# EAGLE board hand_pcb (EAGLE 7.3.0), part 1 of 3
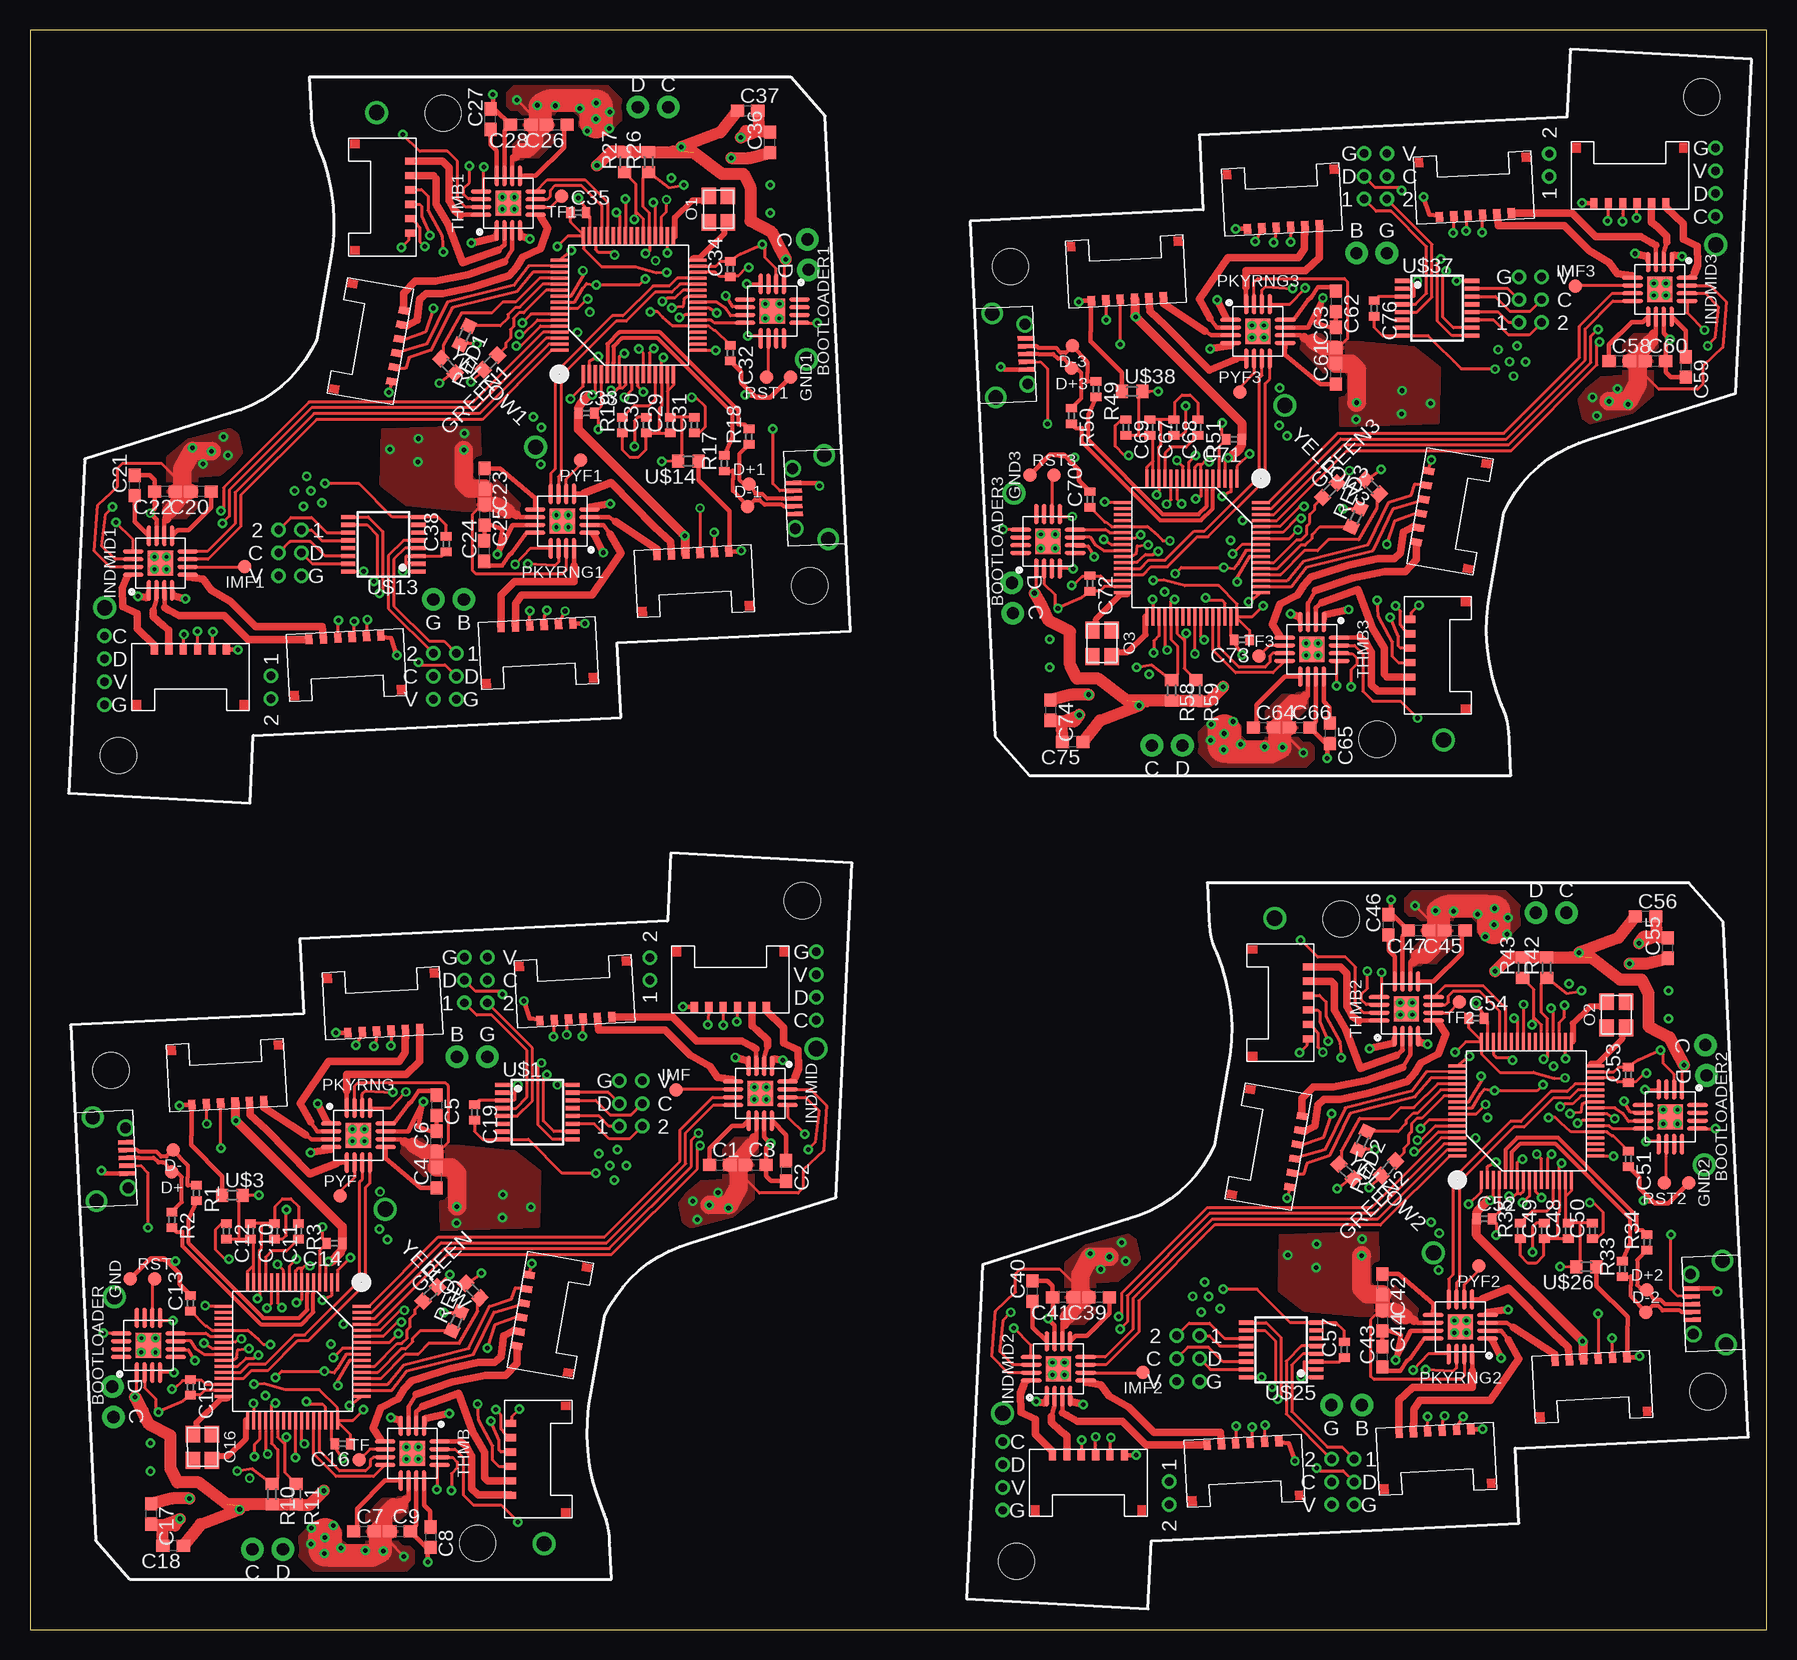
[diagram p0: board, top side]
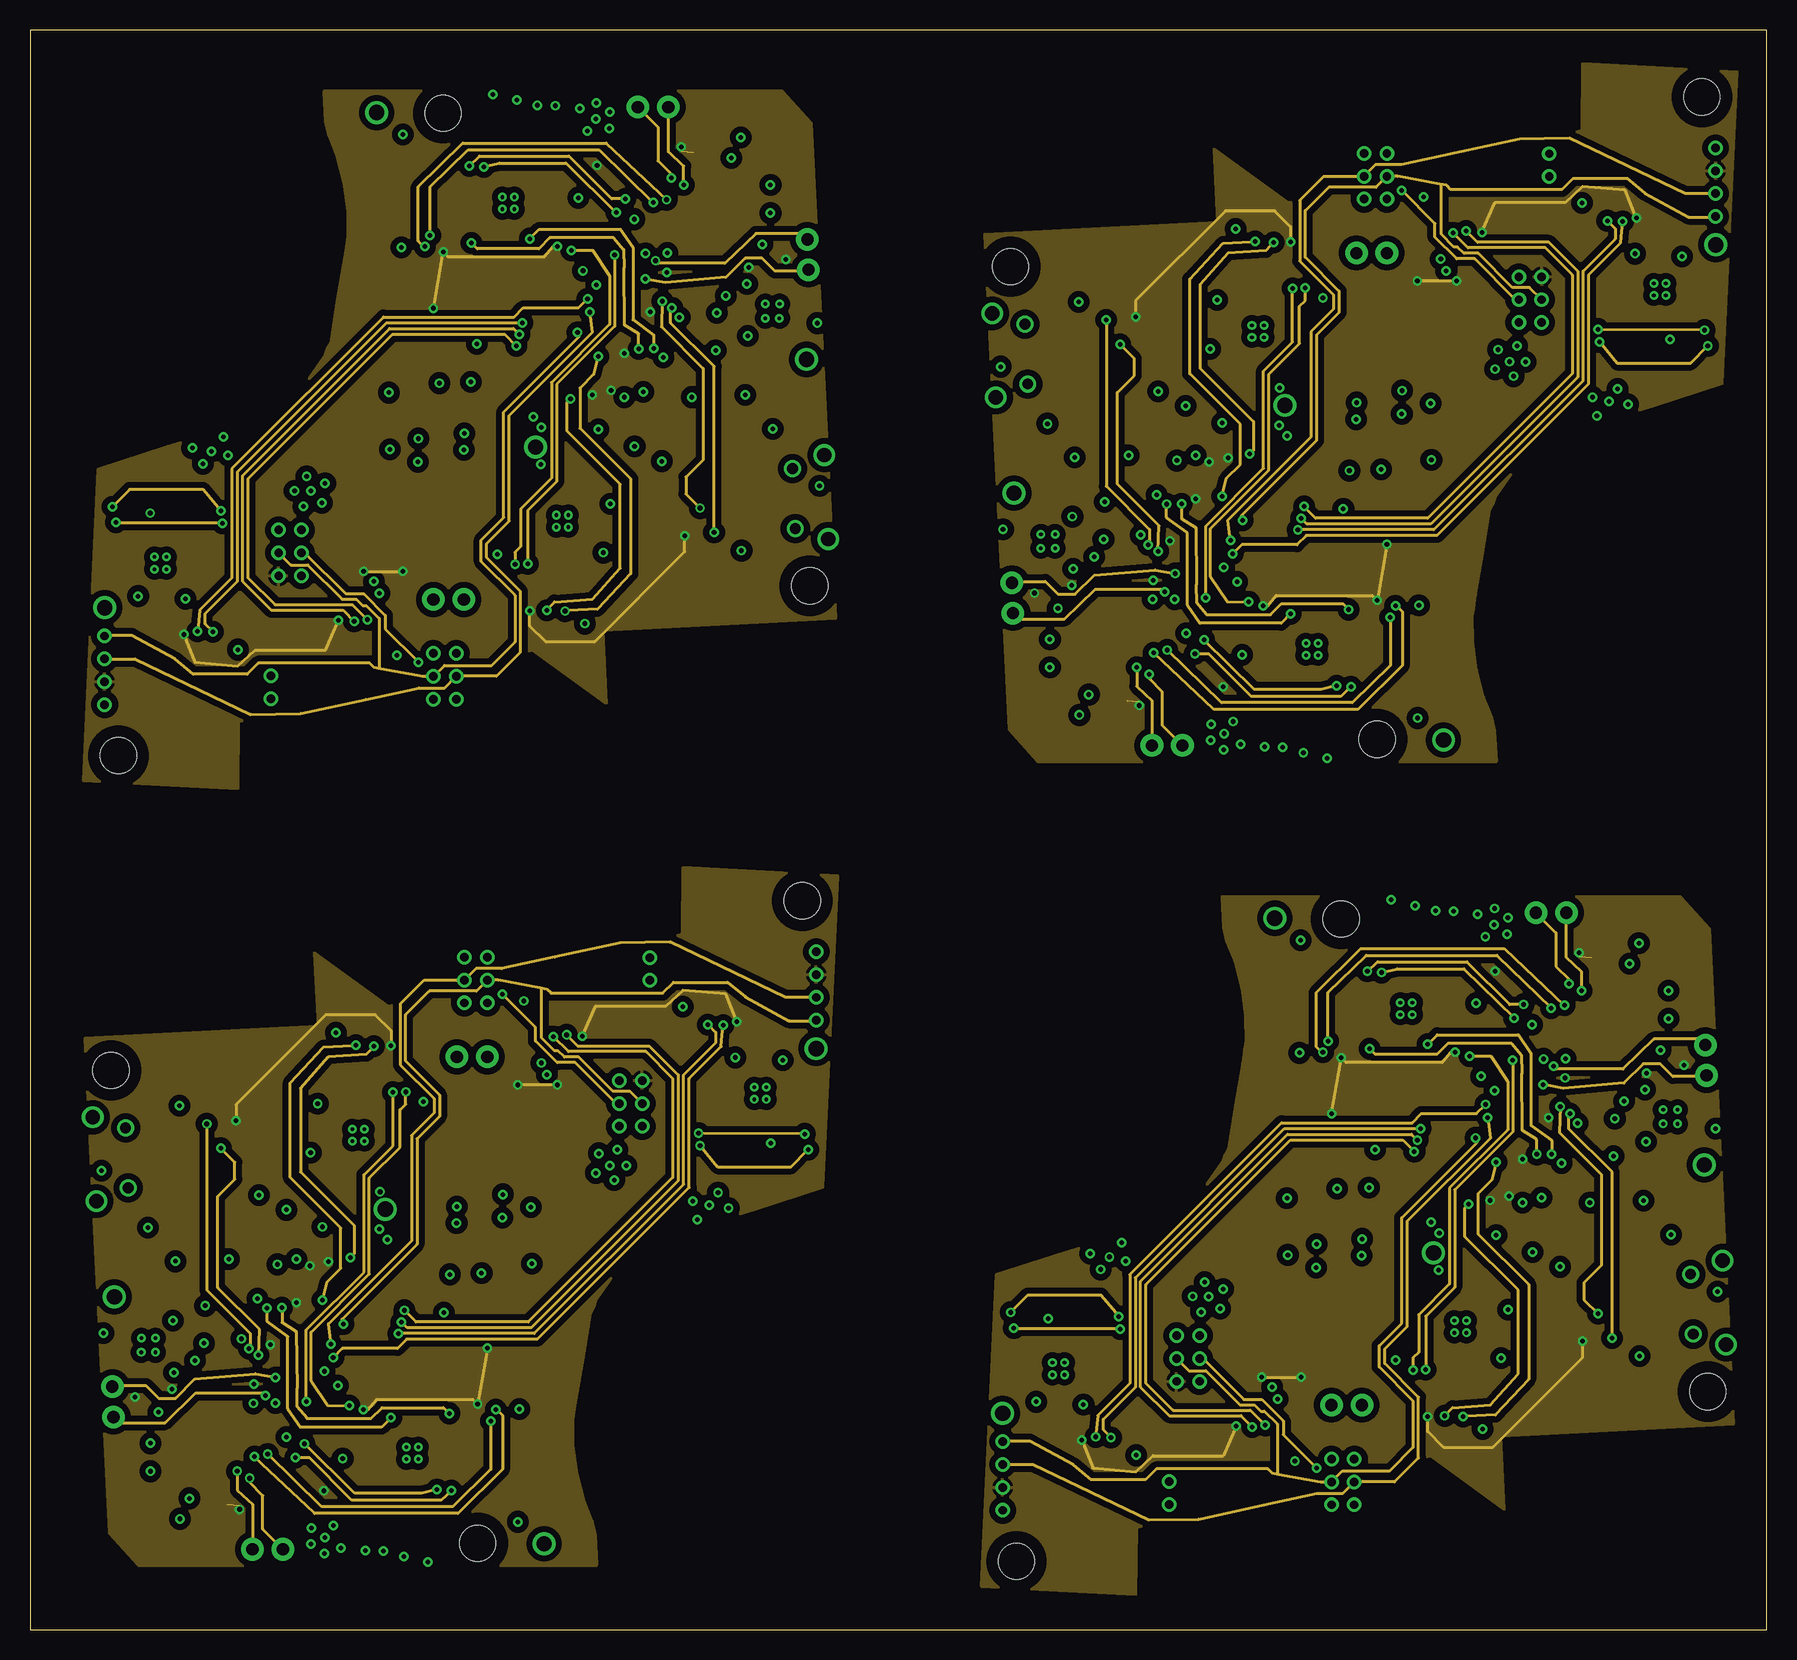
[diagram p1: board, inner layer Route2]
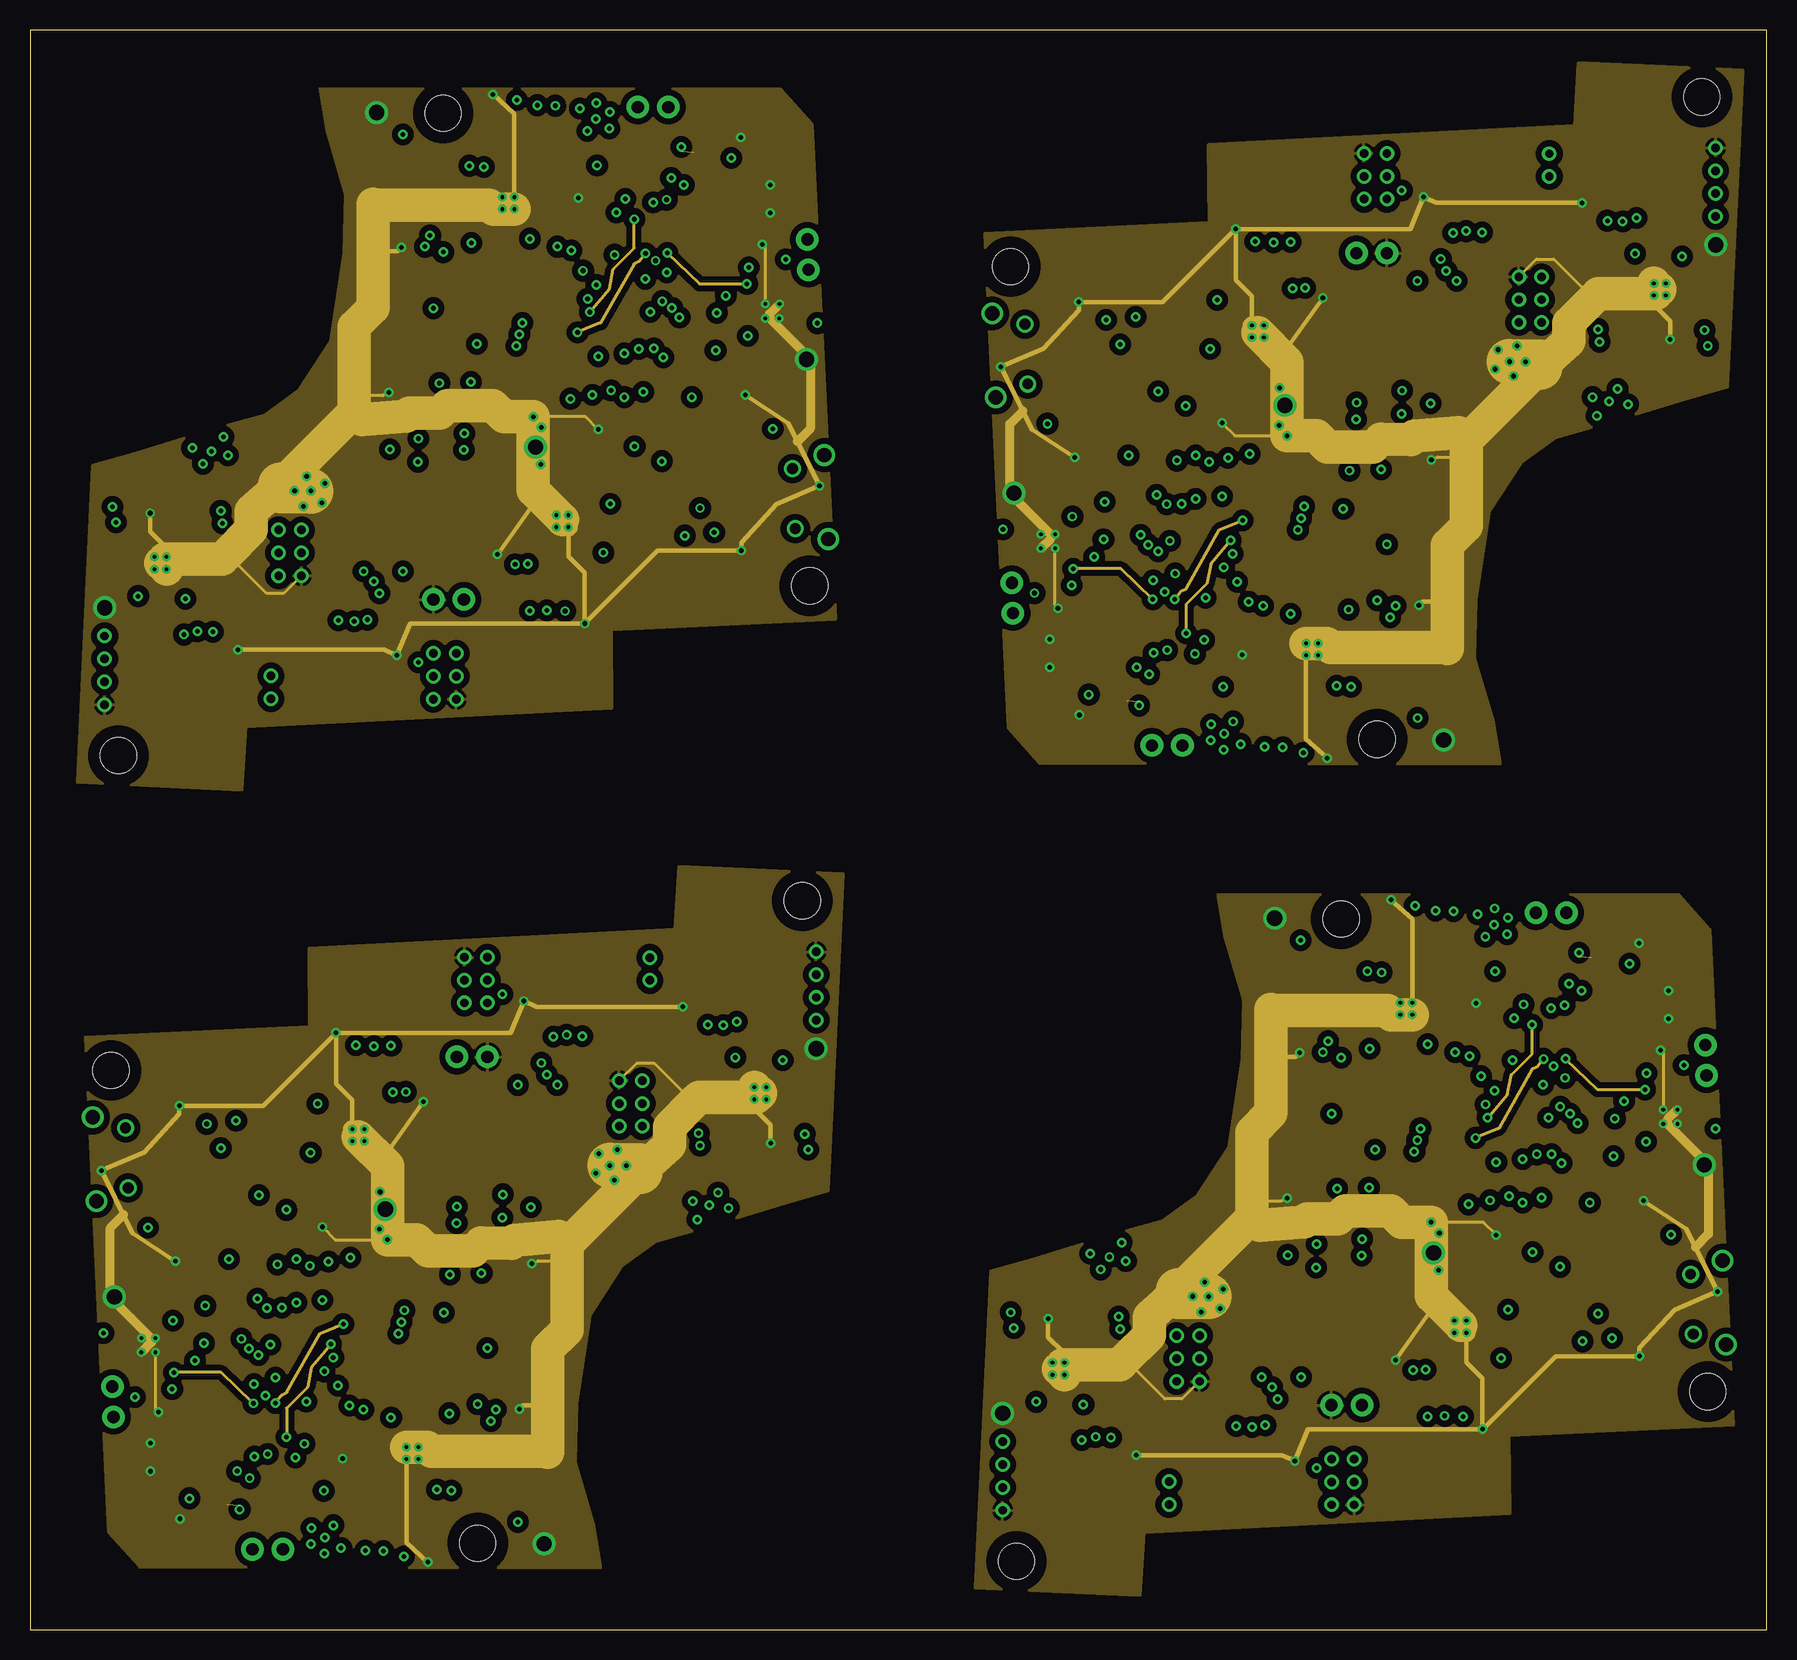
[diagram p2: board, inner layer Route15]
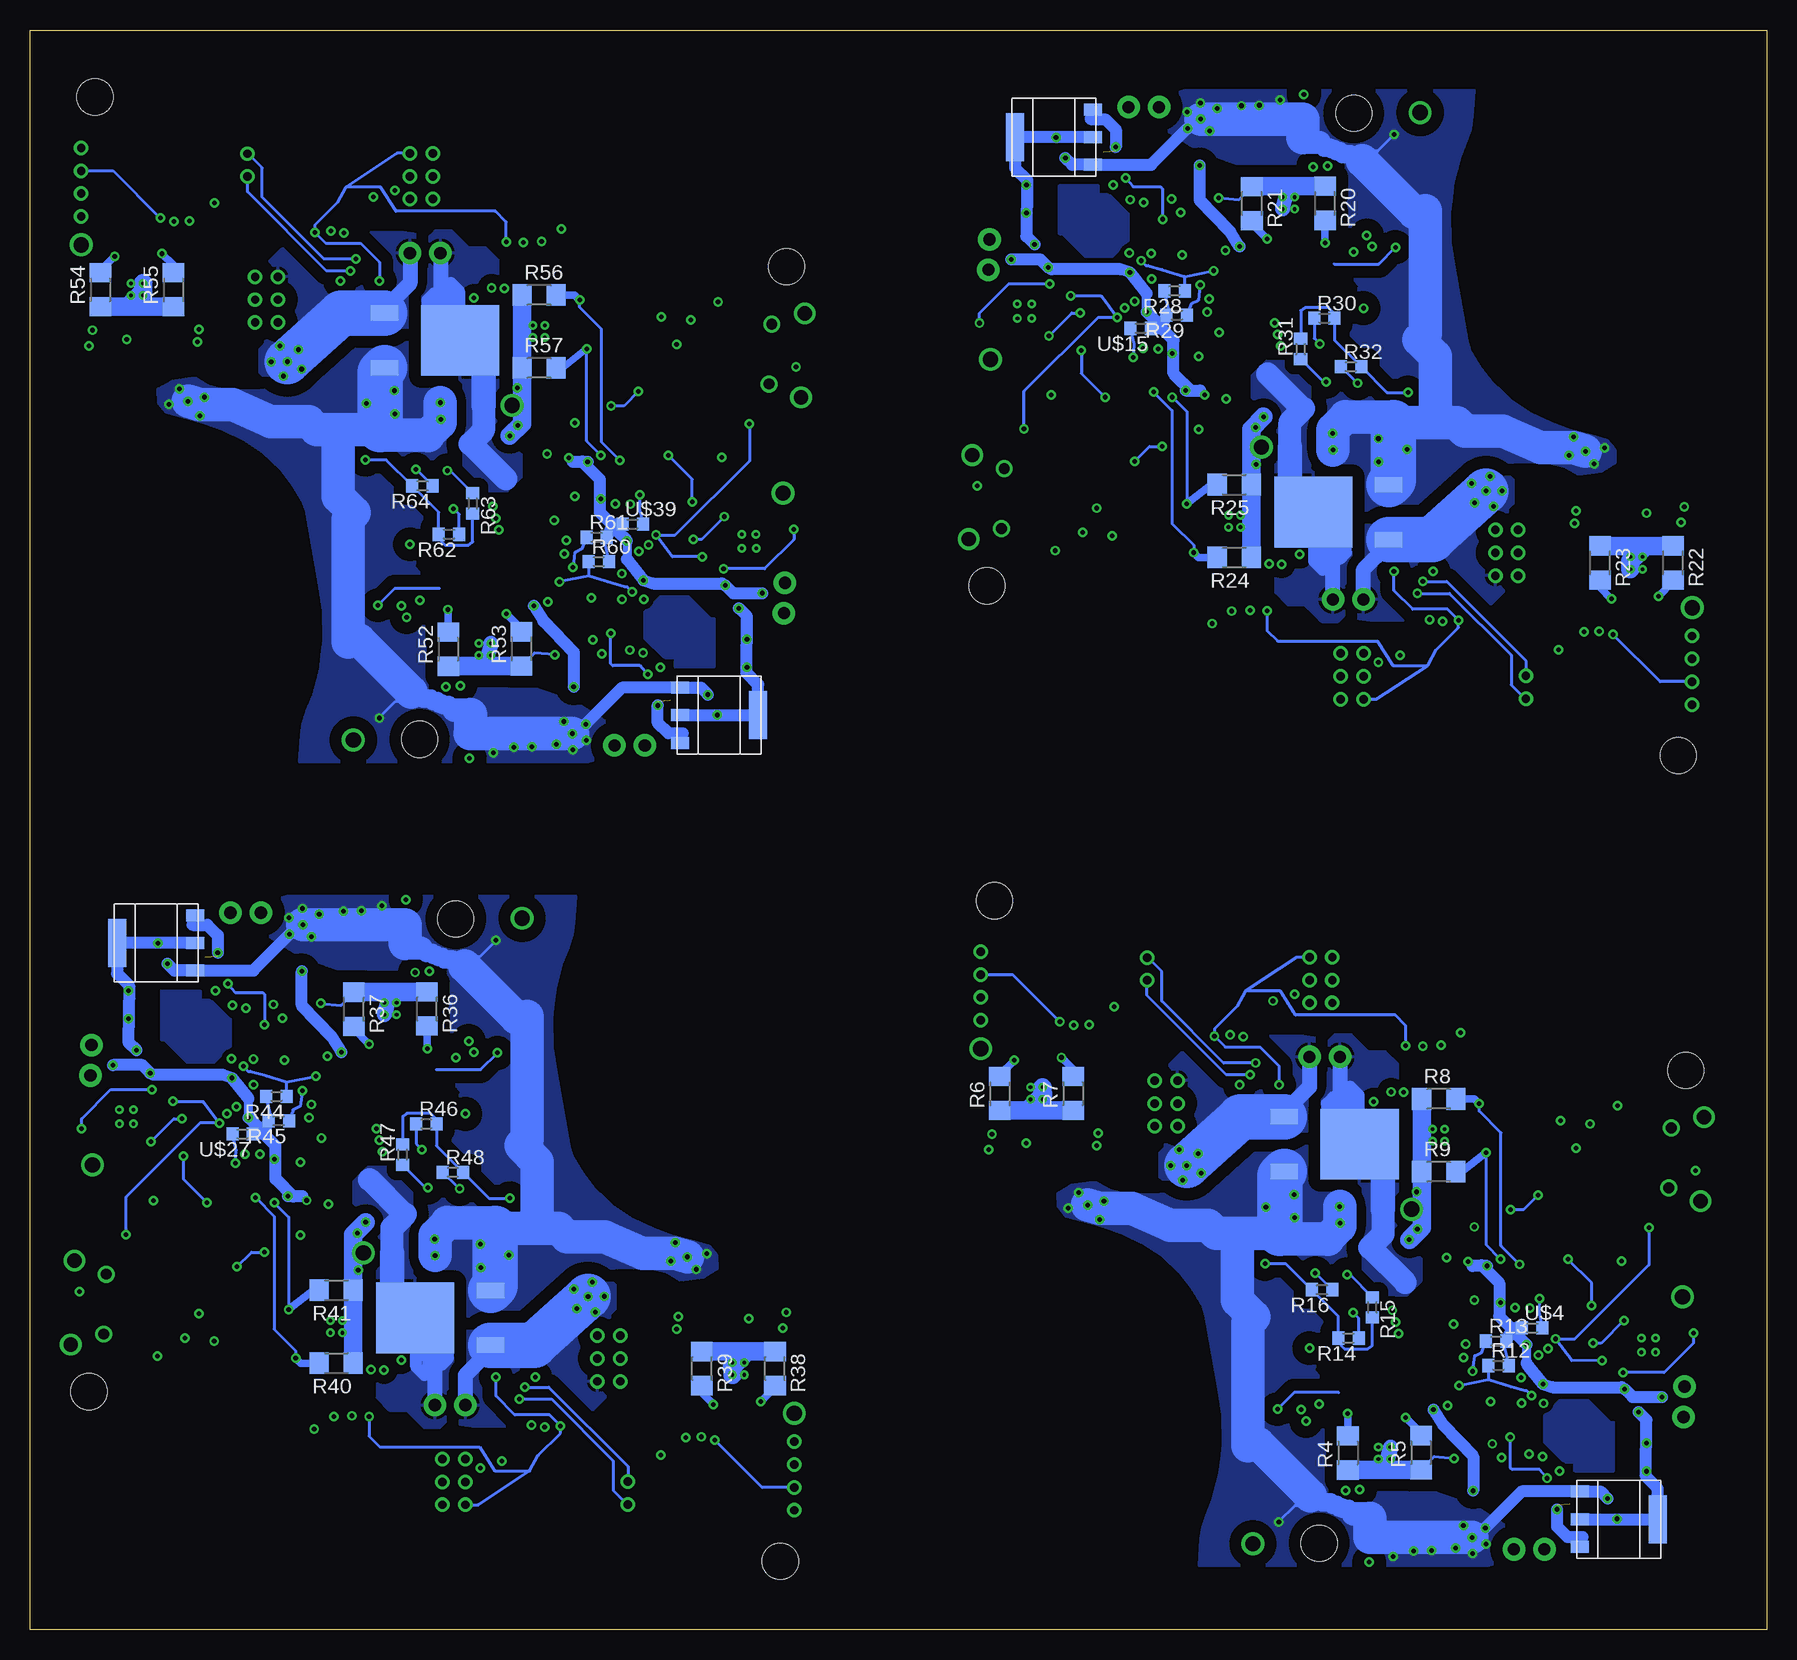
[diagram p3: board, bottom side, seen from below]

Size 144.78 x 133.35 mm. Coordinates in mm from the lower left corner, seen from the top.
Outline: 0,0 144.78,0 144.78,133.35 0,133.35 0,0
Copper layers (1*2*15*16): Top 0.035mm / dielectric 0.2mm / Route2 0.035mm / dielectric 0.2mm / Route15 0.035mm / dielectric 0.2mm / Bottom 0.035mm
Design rules "default *": minimum track width 10mil, minimum drill 15mil, track to track 6mil, track to pad 6mil, pad to pad 6mil, via to via 6mil, smd to smd 6mil, copper to edge 40mil, drill to drill 8mil, minimum pad ring 10mil, minimum via ring 8mil, stop-mask expansion 4mil, vias tented up to drill 0mil, thermal gap 10mil
Net classes: 1 USB: width 0.333 mm, drill 0.333 mm, clearance 0.178 mm; 2 VCC_Pour: clearance 0.762 mm to class 1; 3 GND_Pour: clearance 0.762 mm to class 1
Holes 3 mm at 6.75,46.62 64.38,60.77 37.32,7.22 65.01,87.01 7.38,72.86 34.44,126.41 139.86,19.86 82.23,5.71 109.29,59.26 81.73,113.62 139.36,127.77 112.3,74.22
tKeepout: area 4.6,44.5 to 8.8,48.7; area 62.3,58.7 to 66.5,62.9; area 35.2,5.1 to 39.4,9.3; area 62.9,84.9 to 67.1,89.1; area 5.3,70.8 to 9.5,75; area 32.3,124.3 to 36.5,128.5; area 137.8,17.8 to 142,22; area 80.1,3.6 to 84.3,7.8; area 107.2,57.2 to 111.4,61.4; area 79.6,111.5 to 83.8,115.7; area 137.3,125.7 to 141.5,129.9; area 110.2,72.1 to 114.4,76.3

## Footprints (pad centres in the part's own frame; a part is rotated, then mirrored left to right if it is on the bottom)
WQFN-16 = smd 1.75 x 0.35: 1 -2.275,0.975; 2 -2.275,0.325; 3 -2.275,-0.325; 4 -2.275,-0.975; 9 2.275,-0.975; 10 2.275,-0.325; 11 2.275,0.325; 12 2.275,0.975 | smd 0.35 x 1.75: 5 -0.975,-2.275; 6 -0.325,-2.275; 7 0.325,-2.275; 8 0.975,-2.275; 13 0.975,2.275; 14 0.325,2.275; 15 -0.325,2.275; 16 -0.975,2.275 | smd 2.1 x 2.1: PPAD 0,0
C0603 = smd 1.1 x 1: 1 -0.85,0; 2 0.85,0
C0402 = smd 0.7 x 0.9: 1 -0.65,0; 2 0.65,0
TESTPAD = smd 1.143 x 1.143: P$1 0,0
L0603 = smd 1 x 1.1: 1 -0.85,0; 2 0.85,0
LQFP-64-10-10 = smd 1.5 x 0.254: 1 -5.75,3.75; 2 -5.75,3.25; 3 -5.75,2.75; 4 -5.75,2.25; 5 -5.75,1.75; 6 -5.75,1.25; 7 -5.75,0.75; 8 -5.75,0.25; 9 -5.75,-0.25; 10 -5.75,-0.75; 11 -5.75,-1.25; 12 -5.75,-1.75; 13 -5.75,-2.25; 14 -5.75,-2.75; 15 -5.75,-3.25; 16 -5.75,-3.75; 33 5.75,-3.75; 34 5.75,-3.25; 35 5.75,-2.75; 36 5.75,-2.25; 37 5.75,-1.75; 38 5.75,-1.25; 39 5.75,-0.75; 40 5.75,-0.25; 41 5.75,0.25; 42 5.75,0.75; 43 5.75,1.25; 44 5.75,1.75; 45 5.75,2.25; 46 5.75,2.75; 47 5.75,3.25; 48 5.75,3.75 | smd 0.254 x 1.5: 17 -3.75,-5.75; 18 -3.25,-5.75; 19 -2.75,-5.75; 20 -2.25,-5.75; 21 -1.75,-5.75; 22 -1.25,-5.75; 23 -0.75,-5.75; 24 -0.25,-5.75; 25 0.25,-5.75; 26 0.75,-5.75; 27 1.25,-5.75; 28 1.75,-5.75; 29 2.25,-5.75; 30 2.75,-5.75; 31 3.25,-5.75; 32 3.75,-5.75; 49 3.75,5.75; 50 3.25,5.75; 51 2.75,5.75; 52 2.25,5.75; 53 1.75,5.75; 54 1.25,5.75; 55 0.75,5.75; 56 0.25,5.75; 57 -0.25,5.75; 58 -0.75,5.75; 59 -1.25,5.75; 60 -1.75,5.75; 61 -2.25,5.75; 62 -2.75,5.75; 63 -3.25,5.75; 64 -3.75,5.75
DF57H-6P-TOP = smd 0.6 x 0.85: 1 -3,2.3; 2 -1.8,2.3; 3 -0.6,2.3; 4 0.6,2.3; 5 1.8,2.3; 6 3,2.3
NX3225SA = smd 1.4 x 1.2: 1 -1.1,-0.8; 2 1.1,-0.8; 3 1.1,0.8; 4 -1.1,0.8
R0402 = smd 0.7 x 0.9: 1 -0.65,0; 2 0.65,0
R1206 = smd 1.6 x 1.803: 1 -1.422,0; 2 1.422,0
R0603 = smd 1 x 1.1: 1 -0.85,0; 2 0.85,0
TSSOP16 = smd 0.35 x 1.2: 1 -2.275,-2.925; 2 -1.625,-2.925; 3 -0.975,-2.925; 4 -0.325,-2.925; 5 0.325,-2.925; 6 0.975,-2.925; 7 1.625,-2.925; 8 2.275,-2.925; 9 2.275,2.925; 10 1.625,2.925; 11 0.975,2.925; 12 0.325,2.925; 13 -0.325,2.925; 14 -0.975,2.925; 15 -1.625,2.925; 16 -2.275,2.925
PG-TO-252-3 = smd 1.295 x 2.311: 1 -2.286,-4.191; 3 2.286,-4.191 | smd 5.893 x 6.502: 2 0,2.095
PSENSE = drill 0.7: 1 0,-3.81; 2 1.905,-3.81; C 1.905,-1.905; D 0,-1.905; G 0,0; V 1.905,0
PSENSE2 = drill 0.7: 1 0,0; 2 1.905,0
PSENSE4 = drill 0.7: C 0,-5.715; D 0,-3.81; G 0,0; V 0,-1.905
MIC39100 = smd 1 x 1.5: 1 -2.3,-3.25; 2 0,-3.25; 3 2.3,-3.25 | smd 4 x 1.5: TAB 0,3.25
THRUHOLE2 = drill 1.016 pad 1.88: B -1.27,0; G 1.27,0
THRUHOLEI2C = drill 1.016 pad 1.88: SCL 1.27,0; SDA -1.27,0
10118194-0001LF = smd 0.4 x 1.35: 1 -1.3,2.7; 2 -0.65,2.7; 3 0,2.7; 4 0.65,2.7; 5 1.3,2.7 | drill 0.9 pad 1.4: P$6 -2.5,2.7; P$7 2.5,2.7 | drill 1.2: P$8 -3.5,0; P$9 3.5,0

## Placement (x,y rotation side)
BOOTLOADER  MKL02Z32  [WQFN-16]  9.88,23.72 90 top
BOOTLOADER1  MKL02Z32  [WQFN-16]  61.88,109.91 270 top
BOOTLOADER2  MKL02Z32  [WQFN-16]  136.73,42.76 270 top
BOOTLOADER3  MKL02Z32  [WQFN-16]  84.86,90.72 90 top
C1  0.01  [C0603]  57.49,38.75 0 top
C2  2.2  [C0603]  63.03,38.25 270 top
C3  10  [C0603]  60.51,38.75 0 top
C4  0.01  [C0603]  33.88,37.67 90 top
C5  2.2  [C0603]  33.88,43.71 270 top
C6  10  [C0603]  33.88,40.7 90 top
C7  0.01  [C0603]  27.84,8.19 0 top
C8  2.2  [C0603]  33.38,7.72 270 top
C9  10  [C0603]  30.86,8.2 0 top
C10  2.2  [C0402]  18.38,33.22 270 top
C11  0.1  [C0402]  20.38,33.22 270 top
C12  0.1  [C0402]  16.38,33.22 270 top
C13  0.1  [C0402]  13.38,27.22 90 top
C14  0.1  [C0402]  25.38,32.22 180 top
C15  0.1  [C0402]  13.38,20.22 270 top
C16  0.1  [C0402]  26.05,15.51 180 top
C17  [C0603]  10.08,9.65 270 top
C18  [C0603]  11.94,7.01 180 top
C19  0.1  [C0402]  37.06,43.13 270 top
C20  0.01  [C0603]  14.27,94.88 180 top
C21  2.2  [C0603]  8.72,95.38 90 top
C22  10  [C0603]  11.25,94.87 180 top
C23  0.01  [C0603]  37.88,95.95 270 top
C24  2.2  [C0603]  37.87,89.92 90 top
C25  10  [C0603]  37.88,92.93 270 top
C26  0.01  [C0603]  43.92,125.44 180 top
C27  2.2  [C0603]  38.38,125.91 90 top
C28  10  [C0603]  40.9,125.43 180 top
C29  2.2  [C0402]  53.38,100.41 90 top
C30  0.1  [C0402]  51.38,100.41 90 top
C31  0.1  [C0402]  55.38,100.41 90 top
C32  0.1  [C0402]  58.38,106.41 270 top
C33  0.1  [C0402]  46.38,101.41 0 top
C34  0.1  [C0402]  58.38,113.41 90 top
C35  0.1  [C0402]  45.7,118.12 0 top
C36  [C0603]  61.67,123.98 90 top
C37  [C0603]  59.82,126.62 0 top
C38  0.1  [C0402]  34.7,90.5 90 top
C39  0.01  [C0603]  89.12,27.72 180 top
C40  2.2  [C0603]  83.58,28.22 90 top
C41  10  [C0603]  86.1,27.72 180 top
C42  0.01  [C0603]  112.73,28.8 270 top
C43  2.2  [C0603]  112.73,22.76 90 top
C44  10  [C0603]  112.73,25.77 270 top
C45  0.01  [C0603]  118.77,58.28 180 top
C46  2.2  [C0603]  113.23,58.76 90 top
C47  10  [C0603]  115.75,58.28 180 top
C48  2.2  [C0402]  128.23,33.26 90 top
C49  0.1  [C0402]  126.23,33.26 90 top
C50  0.1  [C0402]  130.23,33.26 90 top
C51  0.1  [C0402]  133.23,39.26 270 top
C52  0.1  [C0402]  121.23,34.26 0 top
C53  0.1  [C0402]  133.23,46.26 90 top
C54  0.1  [C0402]  120.56,50.97 0 top
C55  [C0603]  136.53,56.82 90 top
C56  [C0603]  134.67,59.46 0 top
C57  0.1  [C0402]  109.55,23.34 90 top
C58  0.01  [C0603]  132.47,105.75 0 top
C59  2.2  [C0603]  138.01,105.25 270 top
C60  10  [C0603]  135.49,105.76 0 top
C61  0.01  [C0603]  108.86,104.68 90 top
C62  2.2  [C0603]  108.86,110.72 270 top
C63  10  [C0603]  108.86,107.71 90 top
C64  0.01  [C0603]  102.82,75.2 0 top
C65  2.2  [C0603]  108.36,74.72 270 top
C66  10  [C0603]  105.84,75.2 0 top
C67  2.2  [C0402]  93.36,100.22 270 top
C68  0.1  [C0402]  95.36,100.22 270 top
C69  0.1  [C0402]  91.36,100.22 270 top
C70  0.1  [C0402]  88.36,94.22 90 top
C71  0.1  [C0402]  100.36,99.22 180 top
C72  0.1  [C0402]  88.36,87.22 270 top
C73  0.1  [C0402]  101.03,82.51 180 top
C74  [C0603]  85.06,76.66 270 top
C75  [C0603]  86.92,74.02 180 top
C76  0.1  [C0402]  112.04,110.13 270 top
D+  TESTPAD  [TESTPAD]  11.83,38.15 180 top
D+1  TESTPAD  [TESTPAD]  59.93,95.48 0 top
D+2  TESTPAD  [TESTPAD]  134.78,28.32 0 top
D+3  TESTPAD  [TESTPAD]  86.81,105.15 180 top
D-  TESTPAD  [TESTPAD]  11.92,40.01 180 top
D-1  TESTPAD  [TESTPAD]  59.83,93.62 0 top
D-2  TESTPAD  [TESTPAD]  134.69,26.46 0 top
D-3  TESTPAD  [TESTPAD]  86.9,107.02 180 top
GND  TESTPAD  [TESTPAD]  8.36,29.24 90 top
GND1  TESTPAD  [TESTPAD]  63.4,104.39 270 top
GND2  TESTPAD  [TESTPAD]  138.25,37.24 270 top
GND3  TESTPAD  [TESTPAD]  83.34,96.24 90 top
GREEN  LED0603  [L0603]  33.38,27.99 45 top
GREEN1  LED0603  [L0603]  38.38,105.64 225 top
GREEN2  LED0603  [L0603]  113.23,38.48 225 top
GREEN3  LED0603  [L0603]  108.36,95 45 top
HAND_MICRO  MK20DX256VLH7  [LQFP-64-10-10]  21.88,23.22 270 top
HAND_MICRO1  MK20DX256VLH7  [LQFP-64-10-10]  49.88,110.41 90 top
HAND_MICRO2  MK20DX256VLH7  [LQFP-64-10-10]  124.73,43.26 90 top
HAND_MICRO3  MK20DX256VLH7  [LQFP-64-10-10]  96.86,90.22 270 top
IMF  TESTPAD  [TESTPAD]  53.85,45.01 0 top
IMF1  TESTPAD  [TESTPAD]  17.91,88.62 180 top
IMF2  TESTPAD  [TESTPAD]  92.76,21.46 180 top
IMF3  TESTPAD  [TESTPAD]  128.83,112.01 0 top
INDEX  DF57H-6PTOP  [DF57H-6P-TOP]  58.38,54.22 180 top
INDEX1  DF57H-6PTOP  [DF57H-6P-TOP]  13.38,79.41 0 top
INDEX2  DF57H-6PTOP  [DF57H-6P-TOP]  88.23,12.26 0 top
INDEX3  DF57H-6PTOP  [DF57H-6P-TOP]  133.36,121.22 180 top
INDMID  DRV8833  [WQFN-16]  60.88,44.72 270 top
INDMID1  DRV8833  [WQFN-16]  10.88,88.91 90 top
INDMID2  DRV8833  [WQFN-16]  85.73,21.76 90 top
INDMID3  DRV8833  [WQFN-16]  135.86,111.72 270 top
MIDDLE  DF57H-6PTOP  [DF57H-6P-TOP]  45.38,53.22 183 top
MIDDLE1  DF57H-6PTOP  [DF57H-6P-TOP]  26.38,80.41 3 top
MIDDLE2  DF57H-6PTOP  [DF57H-6P-TOP]  101.23,13.26 3 top
MIDDLE3  DF57H-6PTOP  [DF57H-6P-TOP]  120.36,120.22 183 top
O1  16MHz  [NX3225SA]  57.38,118.41 90 top
O2  16MHz  [NX3225SA]  132.23,51.26 90 top
O3  16MHz  [NX3225SA]  89.36,82.22 270 top
O16  16MHz  [NX3225SA]  14.38,15.22 270 top
PINKY  DF57H-6PTOP  [DF57H-6P-TOP]  16.38,46.22 183 top
PINKY1  DF57H-6PTOP  [DF57H-6P-TOP]  55.38,87.41 3 top
PINKY2  DF57H-6PTOP  [DF57H-6P-TOP]  130.23,20.26 3 top
PINKY3  DF57H-6PTOP  [DF57H-6P-TOP]  91.36,113.22 183 top
PKYRNG  DRV8833  [WQFN-16]  27.38,41.22 0 top
PKYRNG1  DRV8833  [WQFN-16]  44.38,92.41 180 top
PKYRNG2  DRV8833  [WQFN-16]  119.23,25.26 180 top
PKYRNG3  DRV8833  [WQFN-16]  102.36,108.22 0 top
PYF  TESTPAD  [TESTPAD]  25.86,36.14 0 top
PYF1  TESTPAD  [TESTPAD]  45.9,97.49 180 top
PYF2  TESTPAD  [TESTPAD]  120.75,30.33 180 top
PYF3  TESTPAD  [TESTPAD]  100.84,103.15 0 top
R1  33  [R0402]  13.88,36.4 270 top
R2  33  [R0402]  11.83,34.17 270 top
R3  470  [R0402]  22.38,33.22 270 top
R4  0.2  [R1206]  34.92,14.73 90 bottom
R5  0.2  [R1206]  28.83,14.76 90 bottom
R6  0.2  [R1206]  63.93,44.7 90 bottom
R7  0.2  [R1206]  57.84,44.7 90 bottom
R8  0.2  [R1206]  27.36,44.25 0 bottom
R9  0.2  [R1206]  27.36,38.18 0 bottom
R10  1k  [R0603]  20.18,11.3 270 top
R11  1k  [R0603]  22.2,11.3 270 top
R12  1k  [R0603]  22.38,22.02 0 bottom
R13  1k  [R0603]  22.57,24.05 0 bottom
R14  100  [R0603]  34.87,24.31 180 bottom
R15  200  [R0603]  32.89,26.87 270 bottom
R16  200  [R0603]  37.08,28.35 180 bottom
R17  33  [R0402]  57.88,97.23 90 top
R18  33  [R0402]  59.93,99.45 90 top
R19  470  [R0402]  49.38,100.41 90 top
R20  0.2  [R1206]  36.83,118.9 270 bottom
R21  0.2  [R1206]  42.93,118.87 270 bottom
R22  0.2  [R1206]  7.82,88.93 270 bottom
R23  0.2  [R1206]  13.92,88.93 270 bottom
R24  0.2  [R1206]  44.4,89.38 180 bottom
R25  0.2  [R1206]  44.4,95.45 180 bottom
R26  1k  [R0603]  51.57,122.33 90 top
R27  1k  [R0603]  49.56,122.33 90 top
R28  1k  [R0603]  49.38,111.61 180 bottom
R29  1k  [R0603]  49.19,109.58 180 bottom
R30  100  [R0603]  36.88,109.32 0 bottom
R31  200  [R0603]  38.86,106.76 90 bottom
R32  200  [R0603]  34.67,105.28 0 bottom
R33  33  [R0402]  132.73,30.07 90 top
R34  33  [R0402]  134.78,32.3 90 top
R35  470  [R0402]  124.23,33.26 90 top
R36  0.2  [R1206]  111.68,51.74 270 bottom
R37  0.2  [R1206]  117.78,51.71 270 bottom
R38  0.2  [R1206]  82.68,21.77 270 bottom
R39  0.2  [R1206]  88.77,21.77 270 bottom
R40  0.2  [R1206]  119.25,22.23 180 bottom
R41  0.2  [R1206]  119.25,28.3 180 bottom
R42  1k  [R0603]  126.43,55.17 90 top
R43  1k  [R0603]  124.41,55.17 90 top
R44  1k  [R0603]  124.23,44.45 180 bottom
R45  1k  [R0603]  124.04,42.42 180 bottom
R46  100  [R0603]  111.73,42.16 0 bottom
R47  200  [R0603]  113.72,39.6 90 bottom
R48  200  [R0603]  109.52,38.13 0 bottom
R49  33  [R0402]  88.86,103.41 270 top
R50  33  [R0402]  86.81,101.18 270 top
R51  470  [R0402]  97.36,100.22 270 top
R52  0.2  [R1206]  109.91,81.74 90 bottom
R53  0.2  [R1206]  103.81,81.76 90 bottom
R54  0.2  [R1206]  138.91,111.71 90 bottom
R55  0.2  [R1206]  132.82,111.71 90 bottom
R56  0.2  [R1206]  102.34,111.25 0 bottom
R57  0.2  [R1206]  102.34,105.18 0 bottom
R58  1k  [R0603]  95.16,78.31 270 top
R59  1k  [R0603]  97.18,78.31 270 top
R60  1k  [R0603]  97.36,89.03 0 bottom
R61  1k  [R0603]  97.55,91.06 0 bottom
R62  100  [R0603]  109.86,91.31 180 bottom
R63  200  [R0603]  107.87,93.88 270 bottom
R64  200  [R0603]  112.06,95.35 180 bottom
RED  LED0603  [L0603]  35.53,25.7 65 top
RED1  LED0603  [L0603]  36.22,107.92 245 top
RED2  LED0603  [L0603]  111.07,40.77 245 top
RED3  LED0603  [L0603]  110.52,92.71 65 top
RING  DF57H-6PTOP  [DF57H-6P-TOP]  29.38,52.22 183 top
RING1  DF57H-6PTOP  [DF57H-6P-TOP]  42.38,81.41 3 top
RING2  DF57H-6PTOP  [DF57H-6P-TOP]  117.23,14.26 3 top
RING3  DF57H-6PTOP  [DF57H-6P-TOP]  104.36,119.22 183 top
RST  TESTPAD  [TESTPAD]  10.38,29.24 0 top
RST1  TESTPAD  [TESTPAD]  61.38,104.39 180 top
RST2  TESTPAD  [TESTPAD]  136.23,37.24 180 top
RST3  TESTPAD  [TESTPAD]  85.36,96.24 0 top
TF  TESTPAD  [TESTPAD]  27.46,14.15 0 top
TF1  TESTPAD  [TESTPAD]  44.3,119.48 180 top
TF2  TESTPAD  [TESTPAD]  119.15,52.32 180 top
TF3  TESTPAD  [TESTPAD]  102.44,81.15 0 top
THMB  DRV8833  [WQFN-16]  31.88,14.72 270 top
THMB1  DRV8833  [WQFN-16]  39.88,118.91 90 top
THMB2  DRV8833  [WQFN-16]  114.73,51.76 90 top
THMB3  DRV8833  [WQFN-16]  106.86,81.72 270 top
THUMB_A  DF57H-6PTOP  [DF57H-6P-TOP]  42.38,14.22 90 top
THUMB_A1  DF57H-6PTOP  [DF57H-6P-TOP]  29.38,119.41 270 top
THUMB_A2  DF57H-6PTOP  [DF57H-6P-TOP]  104.23,52.26 270 top
THUMB_A3  DF57H-6PTOP  [DF57H-6P-TOP]  117.36,81.22 90 top
THUMB_B  DF57H-6PTOP  [DF57H-6P-TOP]  43.38,26.22 80 top
THUMB_B1  DF57H-6PTOP  [DF57H-6P-TOP]  28.38,107.41 260 top
THUMB_B2  DF57H-6PTOP  [DF57H-6P-TOP]  103.23,40.26 260 top
THUMB_B3  DF57H-6PTOP  [DF57H-6P-TOP]  118.36,93.22 80 top
U$1  TCA9534TSSOP  [TSSOP16]  42.31,43.15 270 top
U$2  SPD15P10PLG  [PG-TO-252-3]  36.04,40.47 270 bottom
U$3  [L0603]  16.88,36.22 0 top
U$4  [L0603]  19.56,25.15 0 bottom
U$5  PSENSE  [PSENSE]  36.22,56.06 0 top
U$6  PSENSE2  [PSENSE2]  51.66,54.13 90 top
U$7  PSENSE  [PSENSE]  49.12,45.77 0 top
U$8  PSENSE4  [PSENSE4]  65.53,56.52 0 top
U$9  MIC391003.3  [MIC39100]  12.34,9.22 270 bottom
U$10  THRUHOLE2  [THRUHOLE2]  36.86,47.75 0 top
U$11  THRUHOLEI2C  [THRUHOLEI2C]  19.81,6.71 180 top
U$12  THRUHOLEI2C  [THRUHOLEI2C]  6.91,19 272 top
U$13  TCA9534TSSOP  [TSSOP16]  29.45,90.48 90 top
U$14  [L0603]  54.88,97.41 180 top
U$15  [L0603]  52.2,108.48 180 bottom
U$16  SPD15P10PLG  [PG-TO-252-3]  35.71,93.15 90 bottom
U$17  PSENSE  [PSENSE]  35.53,77.57 180 top
U$18  PSENSE  [PSENSE]  22.63,87.86 180 top
U$19  PSENSE2  [PSENSE2]  20.09,79.5 270 top
U$20  PSENSE4  [PSENSE4]  6.22,77.11 180 top
U$21  MIC391003.3  [MIC39100]  59.41,124.41 90 bottom
U$22  THRUHOLE2  [THRUHOLE2]  34.9,85.88 180 top
U$23  THRUHOLEI2C  [THRUHOLEI2C]  51.94,126.92 0 top
U$24  THRUHOLEI2C  [THRUHOLEI2C]  64.85,114.63 92 top
U$25  TCA9534TSSOP  [TSSOP16]  104.3,23.32 90 top
U$26  [L0603]  129.73,30.26 180 top
U$27  [L0603]  127.05,41.32 180 bottom
U$28  SPD15P10PLG  [PG-TO-252-3]  110.57,26 90 bottom
U$29  PSENSE  [PSENSE]  110.39,10.41 180 top
U$30  PSENSE  [PSENSE]  97.49,20.7 180 top
U$31  PSENSE2  [PSENSE2]  94.95,12.34 270 top
U$32  PSENSE4  [PSENSE4]  81.08,9.96 180 top
U$33  MIC391003.3  [MIC39100]  134.26,57.25 90 bottom
U$34  THRUHOLE2  [THRUHOLE2]  109.75,18.72 180 top
U$35  THRUHOLEI2C  [THRUHOLEI2C]  126.8,59.77 0 top
U$36  THRUHOLEI2C  [THRUHOLEI2C]  139.7,47.47 92 top
U$37  TCA9534TSSOP  [TSSOP16]  117.29,110.15 270 top
U$38  [L0603]  91.86,103.22 0 top
U$39  [L0603]  94.54,92.16 0 bottom
U$40  SPD15P10PLG  [PG-TO-252-3]  111.02,107.48 270 bottom
U$41  PSENSE  [PSENSE]  111.2,123.06 0 top
U$42  PSENSE  [PSENSE]  124.1,112.78 0 top
U$43  PSENSE2  [PSENSE2]  126.64,121.13 90 top
U$44  PSENSE4  [PSENSE4]  140.51,123.52 0 top
U$45  MIC391003.3  [MIC39100]  87.33,76.23 270 bottom
U$46  THRUHOLE2  [THRUHOLE2]  111.84,114.76 0 top
U$47  THRUHOLEI2C  [THRUHOLEI2C]  94.79,73.71 180 top
U$48  THRUHOLEI2C  [THRUHOLEI2C]  81.89,86 272 top
USB  10118194-0001LF  [10118194-0001LF]  5.38,39.22 272.5 top
USB1  10118194-0001LF  [10118194-0001LF]  66.38,94.41 92.5 top
USB2  10118194-0001LF  [10118194-0001LF]  141.23,27.26 92.5 top
USB3  10118194-0001LF  [10118194-0001LF]  80.36,106.22 272.5 top
YELLOW  LED0603  [L0603]  36.91,28.27 135 top
YELLOW1  LED0603  [L0603]  34.85,105.36 315 top
YELLOW2  LED0603  [L0603]  109.7,38.2 315 top
YELLOW3  LED0603  [L0603]  111.89,95.28 135 top

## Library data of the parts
BOOTLOADER BOOTLOADER1-BOOTLOADER3 D+ D+1-D+3 D- D-1-D-3 GND GND1-GND3 GREEN GREEN1-GREEN3 HAND_MICRO HAND_MICRO1-HAND_MICRO3 IMF IMF1-IMF3 INDEX INDEX1-INDEX3 INDMID INDMID1-INDMID3 MIDDLE MIDDLE1-MIDDLE3 O1-O3 O16 PINKY PINKY1-PINKY3 PKYRNG PKYRNG1-PKYRNG3 PYF PYF1-PYF3 RED RED1-RED3 RING RING1-RING3 RST RST1-RST3 TF TF1-TF3 THMB THMB1-THMB3 THUMB_A THUMB_A1-THUMB_A3 THUMB_B THUMB_B1-THUMB_B3 U$1-U$48 USB USB1-USB3 YELLOW YELLOW1-YELLOW3 = 445-eagle-lib
C1-C76 R1-R64 = rcl

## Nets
+3V1: BOOTLOADER1.1 C32.1 C33.1 C34.1 C35.1 C37.1 C38.1 HAND_MICRO1.3 HAND_MICRO1.7 HAND_MICRO1.8 HAND_MICRO1.21 HAND_MICRO1.30 HAND_MICRO1.48 INDEX1.3 MIDDLE1.3 PINKY1.3 R26.2 R27.2 R28.2 R29.2 RING1.3 THUMB_A1.3 THUMB_B1.3 U$13.1 U$13.2 U$13.3 U$13.16 U$15.1 U$17.V U$18.V U$20.V U$21.3
+3V2: BOOTLOADER2.1 C51.1 C52.1 C53.1 C54.1 C56.1 C57.1 HAND_MICRO2.3 HAND_MICRO2.7 HAND_MICRO2.8 HAND_MICRO2.21 HAND_MICRO2.30 HAND_MICRO2.48 INDEX2.3 MIDDLE2.3 PINKY2.3 R42.2 R43.2 R44.2 R45.2 RING2.3 THUMB_A2.3 THUMB_B2.3 U$25.1 U$25.2 U$25.3 U$25.16 U$27.1 U$29.V U$30.V U$32.V U$33.3
+3V3: BOOTLOADER.1 C13.1 C14.1 C15.1 C16.1 C18.1 C19.1 HAND_MICRO.3 HAND_MICRO.7 HAND_MICRO.8 HAND_MICRO.21 HAND_MICRO.30 HAND_MICRO.48 INDEX.3 MIDDLE.3 PINKY.3 R10.2 R11.2 R12.2 R13.2 RING.3 THUMB_A.3 THUMB_B.3 U$1.1 U$1.2 U$1.3 U$1.16 U$4.1 U$5.V U$7.V U$8.V U$9.3
+3V4: BOOTLOADER3.1 C70.1 C71.1 C72.1 C73.1 C75.1 C76.1 HAND_MICRO3.3 HAND_MICRO3.7 HAND_MICRO3.8 HAND_MICRO3.21 HAND_MICRO3.30 HAND_MICRO3.48 INDEX3.3 MIDDLE3.3 PINKY3.3 R58.2 R59.2 R60.2 R61.2 RING3.3 THUMB_A3.3 THUMB_B3.3 U$37.1 U$37.2 U$37.3 U$37.16 U$39.1 U$41.V U$42.V U$44.V U$45.3
+5V: C1.2 C3.1 C4.2 C6.1 C7.2 C9.1 C17.1 INDMID.10 INDMID.15 PKYRNG.10 PKYRNG.15 THMB.10 THMB.15 U$2.3 U$9.1
+5V1: C20.2 C22.1 C23.2 C25.1 C26.2 C28.1 C36.1 INDMID1.10 INDMID1.15 PKYRNG1.10 PKYRNG1.15 THMB1.10 THMB1.15 U$16.3 U$21.1
+5V2: C39.2 C41.1 C42.2 C44.1 C45.2 C47.1 C55.1 INDMID2.10 INDMID2.15 PKYRNG2.10 PKYRNG2.15 THMB2.10 THMB2.15 U$28.3 U$33.1
+5V3: C58.2 C60.1 C61.2 C63.1 C64.2 C66.1 C74.1 INDMID3.10 INDMID3.15 PKYRNG3.10 PKYRNG3.15 THMB3.10 THMB3.15 U$40.3 U$45.1
EN1: U$1.4 U$5.1
EN2: U$1.5 U$5.2
EN3: U$1.12 U$7.1
EN4: U$1.11 U$7.2
EN5: U$1.10 U$6.1
EN6: U$1.9 U$6.2
EN7: U$13.4 U$17.1
EN8: U$13.5 U$17.2
EN9: U$13.9 U$19.2
EN10: U$13.12 U$18.1
EN11: U$13.11 U$18.2
EN12: U$13.10 U$19.1
EN13: U$25.4 U$29.1
EN14: U$25.5 U$29.2
EN15: U$25.9 U$31.2
EN16: U$25.12 U$30.1
EN17: U$25.11 U$30.2
EN18: U$25.10 U$31.1
EN19: U$37.4 U$41.1
EN20: U$37.5 U$41.2
EN21: U$37.9 U$43.2
EN22: U$37.12 U$42.1
EN23: U$37.11 U$42.2
EN24: U$37.10 U$43.1
GND: BOOTLOADER.2 BOOTLOADER.PPAD C2.2 C3.2 C5.2 C6.2 C8.2 C9.2 C13.2 C14.2 C15.2 C16.2 C17.2 C18.2 C19.2 GND.P$1 HAND_MICRO.4 HAND_MICRO.31 HAND_MICRO.47 INDEX.6 INDMID.11 INDMID.PPAD MIDDLE.6 PINKY.6 PKYRNG.11 PKYRNG.PPAD R4.1 R5.1 R6.1 R7.1 R8.1 R9.1 R14.2 R15.2 R16.2 RING.6 THMB.11 THMB.PPAD THUMB_A.6 THUMB_B.6 U$1.8 U$2.1 U$3.1 U$5.G U$7.G U$8.G U$9.2 U$9.TAB U$10.G USB.5
GND1: BOOTLOADER1.2 BOOTLOADER1.PPAD C21.2 C22.2 C24.2 C25.2 C27.2 C28.2 C32.2 C33.2 C34.2 C35.2 C36.2 C37.2 C38.2 GND1.P$1 HAND_MICRO1.4 HAND_MICRO1.31 HAND_MICRO1.47 INDEX1.6 INDMID1.11 INDMID1.PPAD MIDDLE1.6 PINKY1.6 PKYRNG1.11 PKYRNG1.PPAD R20.1 R21.1 R22.1 R23.1 R24.1 R25.1 R30.2 R31.2 R32.2 RING1.6 THMB1.11 THMB1.PPAD THUMB_A1.6 THUMB_B1.6 U$13.8 U$14.1 U$16.1 U$17.G U$18.G U$20.G U$21.2 U$21.TAB U$22.G USB1.5
GND2: BOOTLOADER2.2 BOOTLOADER2.PPAD C40.2 C41.2 C43.2 C44.2 C46.2 C47.2 C51.2 C52.2 C53.2 C54.2 C55.2 C56.2 C57.2 GND2.P$1 HAND_MICRO2.4 HAND_MICRO2.31 HAND_MICRO2.47 INDEX2.6 INDMID2.11 INDMID2.PPAD MIDDLE2.6 PINKY2.6 PKYRNG2.11 PKYRNG2.PPAD R36.1 R37.1 R38.1 R39.1 R40.1 R41.1 R46.2 R47.2 R48.2 RING2.6 THMB2.11 THMB2.PPAD THUMB_A2.6 THUMB_B2.6 U$25.8 U$26.1 U$28.1 U$29.G U$30.G U$32.G U$33.2 U$33.TAB U$34.G USB2.5
GND3: BOOTLOADER3.2 BOOTLOADER3.PPAD C59.2 C60.2 C62.2 C63.2 C65.2 C66.2 C70.2 C71.2 C72.2 C73.2 C74.2 C75.2 C76.2 GND3.P$1 HAND_MICRO3.4 HAND_MICRO3.31 HAND_MICRO3.47 INDEX3.6 INDMID3.11 INDMID3.PPAD MIDDLE3.6 PINKY3.6 PKYRNG3.11 PKYRNG3.PPAD R52.1 R53.1 R54.1 R55.1 R56.1 R57.1 R62.2 R63.2 R64.2 RING3.6 THMB3.11 THMB3.PPAD THUMB_A3.6 THUMB_B3.6 U$37.8 U$38.1 U$40.1 U$41.G U$42.G U$44.G U$45.2 U$45.TAB U$46.G USB3.5
IDX1: INDEX.1 INDMID.16
IDX2: INDEX.2 INDMID.2
IDX3: INDEX1.1 INDMID1.16
IDX4: INDEX1.2 INDMID1.2
IDX5: INDEX2.1 INDMID2.16
IDX6: INDEX2.2 INDMID2.2
IDX7: INDEX3.1 INDMID3.16
IDX8: INDEX3.2 INDMID3.2
IDXENC1: HAND_MICRO.58 INDEX.5
IDXENC2: HAND_MICRO.57 INDEX.4
IDXENC3: HAND_MICRO1.57 INDEX1.4
IDXENC4: HAND_MICRO1.58 INDEX1.5
IDXENC5: HAND_MICRO2.57 INDEX2.4
IDXENC6: HAND_MICRO2.58 INDEX2.5
IDXENC7: HAND_MICRO3.57 INDEX3.4
IDXENC8: HAND_MICRO3.58 INDEX3.5
IDXISEN: INDMID.1 R6.2
IDXISEN1: INDMID1.1 R22.2
IDXISEN2: INDMID2.1 R38.2
IDXISEN3: INDMID3.1 R54.2
IDXPWM1: HAND_MICRO.61 INDMID.14
IDXPWM2: HAND_MICRO.62 INDMID.13
IDXPWM3: HAND_MICRO1.62 INDMID1.13
IDXPWM4: HAND_MICRO1.61 INDMID1.14
IDXPWM5: HAND_MICRO2.62 INDMID2.13
IDXPWM6: HAND_MICRO2.61 INDMID2.14
IDXPWM7: HAND_MICRO3.62 INDMID3.13
IDXPWM8: HAND_MICRO3.61 INDMID3.14
LED0: HAND_MICRO.53 RED.1
LED1: GREEN.1 HAND_MICRO.54
LED2: HAND_MICRO.52 YELLOW.1
LED3: HAND_MICRO1.53 RED1.1
LED4: GREEN1.1 HAND_MICRO1.54
LED5: HAND_MICRO1.52 YELLOW1.1
LED6: HAND_MICRO2.53 RED2.1
LED7: GREEN2.1 HAND_MICRO2.54
LED8: HAND_MICRO2.52 YELLOW2.1
LED9: HAND_MICRO3.53 RED3.1
LED10: GREEN3.1 HAND_MICRO3.54
LED11: HAND_MICRO3.52 YELLOW3.1
MID1: INDMID.5 MIDDLE.2
MID2: INDMID.3 MIDDLE.1
MID3: INDMID1.3 MIDDLE1.1
MID4: INDMID1.5 MIDDLE1.2
MID5: INDMID2.3 MIDDLE2.1
MID6: INDMID2.5 MIDDLE2.2
MID7: INDMID3.3 MIDDLE3.1
MID8: INDMID3.5 MIDDLE3.2
MIDENC1: HAND_MICRO.60 MIDDLE.5
MIDENC2: HAND_MICRO.59 MIDDLE.4
MIDENC3: HAND_MICRO1.59 MIDDLE1.4
MIDENC4: HAND_MICRO1.60 MIDDLE1.5
MIDENC5: HAND_MICRO2.59 MIDDLE2.4
MIDENC6: HAND_MICRO2.60 MIDDLE2.5
MIDENC7: HAND_MICRO3.59 MIDDLE3.4
MIDENC8: HAND_MICRO3.60 MIDDLE3.5
MIDISEN: INDMID.4 R7.2
MIDISEN1: INDMID1.4 R23.2
MIDISEN2: INDMID2.4 R39.2
MIDISEN3: INDMID3.4 R55.2
MIDPWM1: HAND_MICRO.64 INDMID.7
MIDPWM2: HAND_MICRO.63 INDMID.8
MIDPWM3: HAND_MICRO1.63 INDMID1.8
MIDPWM4: HAND_MICRO1.64 INDMID1.7
MIDPWM5: HAND_MICRO2.63 INDMID2.8
MIDPWM6: HAND_MICRO2.64 INDMID2.7
MIDPWM7: HAND_MICRO3.63 INDMID3.8
MIDPWM8: HAND_MICRO3.64 INDMID3.7
N$1: R14.1 RED.2
N$2: GREEN.2 R15.1
N$3: R16.1 YELLOW.2
N$4: IMF.P$1 INDMID.6
N$5: PKYRNG.6 PYF.P$1
N$6: TF.P$1 THMB.6
N$7: BOOTLOADER1.7 HAND_MICRO1.25
N$8: BOOTLOADER1.8 HAND_MICRO1.22
N$9: BOOTLOADER1.9 HAND_MICRO1.24
N$10: BOOTLOADER1.4 BOOTLOADER1.13 HAND_MICRO1.34
N$11: C29.2 C30.2 C31.2 HAND_MICRO1.15 HAND_MICRO1.16 U$14.2
N$12: C20.1 INDMID1.9
N$13: BOOTLOADER.7 HAND_MICRO.25
N$14: BOOTLOADER.8 HAND_MICRO.22
N$15: BOOTLOADER.9 HAND_MICRO.24
N$16: C23.1 PKYRNG1.9
N$17: BOOTLOADER.4 BOOTLOADER.13 HAND_MICRO.34
N$18: C10.2 C11.2 C12.2 HAND_MICRO.15 HAND_MICRO.16 U$3.2
N$19: C26.1 THMB1.9
N$20: C27.1 THMB1.12
N$21: C1.1 INDMID.9
N$22: C4.1 PKYRNG.9
N$23: C7.1 THMB.9
N$24: HAND_MICRO.33 O16.3
N$25: C8.1 THMB.12
N$26: C5.1 PKYRNG.12
N$27: C2.1 INDMID.12
N$28: HAND_MICRO.32 O16.1
N$29: C24.1 PKYRNG1.12
N$30: C21.1 INDMID1.12
N$31: BOOTLOADER.10 RST.P$1
N$32: HAND_MICRO.13 R3.2
N$33: C10.1 C11.1 HAND_MICRO.14 R3.1 U$4.2
N$34: C12.1 HAND_MICRO.17
N$35: BOOTLOADER.6 HAND_MICRO.23 USB.4
N$36: HAND_MICRO1.33 O1.3
N$37: HAND_MICRO1.32 O1.1
N$38: BOOTLOADER1.10 RST1.P$1
N$39: HAND_MICRO1.13 R19.2
N$40: C29.1 C30.1 HAND_MICRO1.14 R19.1 U$15.2
N$41: C31.1 HAND_MICRO1.17
N$42: BOOTLOADER1.6 HAND_MICRO1.23 USB1.4
N$43: R30.1 RED1.2
N$44: GREEN1.2 R31.1
N$45: R32.1 YELLOW1.2
N$46: IMF1.P$1 INDMID1.6
N$47: PKYRNG1.6 PYF1.P$1
N$48: TF1.P$1 THMB1.6
N$49: BOOTLOADER2.7 HAND_MICRO2.25
N$50: BOOTLOADER2.8 HAND_MICRO2.22
N$51: BOOTLOADER2.9 HAND_MICRO2.24
N$52: BOOTLOADER2.4 BOOTLOADER2.13 HAND_MICRO2.34
N$53: C48.2 C49.2 C50.2 HAND_MICRO2.15 HAND_MICRO2.16 U$26.2
N$54: C39.1 INDMID2.9
N$55: C42.1 PKYRNG2.9
N$56: C45.1 THMB2.9
N$57: C46.1 THMB2.12
N$58: C43.1 PKYRNG2.12
N$59: C40.1 INDMID2.12
N$60: HAND_MICRO2.33 O2.3
N$61: HAND_MICRO2.32 O2.1
N$62: BOOTLOADER2.10 RST2.P$1
N$63: HAND_MICRO2.13 R35.2
N$64: C48.1 C49.1 HAND_MICRO2.14 R35.1 U$27.2
N$65: C50.1 HAND_MICRO2.17
N$66: BOOTLOADER2.6 HAND_MICRO2.23 USB2.4
N$67: R46.1 RED2.2
N$68: GREEN2.2 R47.1
N$69: R48.1 YELLOW2.2
N$70: IMF2.P$1 INDMID2.6
N$71: PKYRNG2.6 PYF2.P$1
N$72: TF2.P$1 THMB2.6
N$73: BOOTLOADER3.7 HAND_MICRO3.25
N$74: BOOTLOADER3.8 HAND_MICRO3.22
N$75: BOOTLOADER3.9 HAND_MICRO3.24
N$76: BOOTLOADER3.4 BOOTLOADER3.13 HAND_MICRO3.34
N$77: C67.2 C68.2 C69.2 HAND_MICRO3.15 HAND_MICRO3.16 U$38.2
N$78: C58.1 INDMID3.9
N$79: C61.1 PKYRNG3.9
N$80: C64.1 THMB3.9
N$81: C65.1 THMB3.12
N$82: C62.1 PKYRNG3.12
N$83: C59.1 INDMID3.12
N$84: HAND_MICRO3.33 O3.3
N$85: HAND_MICRO3.32 O3.1
N$86: BOOTLOADER3.10 RST3.P$1
N$87: HAND_MICRO3.13 R51.2
N$88: C67.1 C68.1 HAND_MICRO3.14 R51.1 U$39.2
N$89: C69.1 HAND_MICRO3.17
N$90: BOOTLOADER3.6 HAND_MICRO3.23 USB3.4
N$91: R62.1 RED3.2
N$92: GREEN3.2 R63.1
N$93: R64.1 YELLOW3.2
N$94: IMF3.P$1 INDMID3.6
N$95: PKYRNG3.6 PYF3.P$1
N$96: TF3.P$1 THMB3.6
PKY1: PINKY.2 PKYRNG.5
PKY2: PINKY.1 PKYRNG.3
PKY3: PINKY1.2 PKYRNG1.5
PKY4: PINKY1.1 PKYRNG1.3
PKY5: PINKY2.2 PKYRNG2.5
PKY6: PINKY2.1 PKYRNG2.3
PKY7: PINKY3.2 PKYRNG3.5
PKY8: PINKY3.1 PKYRNG3.3
PKYENC1: HAND_MICRO.26 PINKY.5
PKYENC2: HAND_MICRO.27 PINKY.4
PKYENC3: HAND_MICRO1.26 PINKY1.5
PKYENC4: HAND_MICRO1.27 PINKY1.4
PKYENC5: HAND_MICRO2.26 PINKY2.5
PKYENC6: HAND_MICRO2.27 PINKY2.4
PKYENC7: HAND_MICRO3.26 PINKY3.5
PKYENC8: HAND_MICRO3.27 PINKY3.4
PKYISEN: HAND_MICRO.9 PKYRNG.4 R9.2
PKYISEN1: HAND_MICRO1.9 PKYRNG1.4 R25.2
PKYISEN2: HAND_MICRO2.9 PKYRNG2.4 R41.2
PKYISEN3: HAND_MICRO3.9 PKYRNG3.4 R57.2
PKYPWM1: HAND_MICRO.28 PKYRNG.7
PKYPWM2: HAND_MICRO.29 PKYRNG.8
PKYPWM3: HAND_MICRO1.29 PKYRNG1.8
PKYPWM4: HAND_MICRO1.28 PKYRNG1.7
PKYPWM5: HAND_MICRO2.29 PKYRNG2.8
PKYPWM6: HAND_MICRO2.28 PKYRNG2.7
PKYPWM7: HAND_MICRO3.29 PKYRNG3.8
PKYPWM8: HAND_MICRO3.28 PKYRNG3.7
RNG1: PKYRNG.16 RING.1
RNG2: PKYRNG.2 RING.2
RNG3: PKYRNG1.16 RING1.1
RNG4: PKYRNG1.2 RING1.2
RNG5: PKYRNG2.16 RING2.1
RNG6: PKYRNG2.2 RING2.2
RNG7: PKYRNG3.16 RING3.1
RNG8: PKYRNG3.2 RING3.2
RNGENC1: HAND_MICRO.2 RING.5
RNGENC2: HAND_MICRO.1 RING.4
RNGENC3: HAND_MICRO1.1 RING1.4
RNGENC4: HAND_MICRO1.2 RING1.5
RNGENC5: HAND_MICRO2.1 RING2.4
RNGENC6: HAND_MICRO2.2 RING2.5
RNGENC7: HAND_MICRO3.1 RING3.4
RNGENC8: HAND_MICRO3.2 RING3.5
RNGISEN: HAND_MICRO.10 PKYRNG.1 R8.2
RNGISEN1: HAND_MICRO1.10 PKYRNG1.1 R24.2
RNGISEN2: HAND_MICRO2.10 PKYRNG2.1 R40.2
RNGISEN3: HAND_MICRO3.10 PKYRNG3.1 R56.2
RNGPWM1: HAND_MICRO.46 PKYRNG.14
RNGPWM2: HAND_MICRO.49 PKYRNG.13
RNGPWM3: HAND_MICRO1.49 PKYRNG1.13
RNGPWM4: HAND_MICRO1.46 PKYRNG1.14
RNGPWM5: HAND_MICRO2.49 PKYRNG2.13
RNGPWM6: HAND_MICRO2.46 PKYRNG2.14
RNGPWM7: HAND_MICRO3.49 PKYRNG3.13
RNGPWM8: HAND_MICRO3.46 PKYRNG3.14
SCL0: HAND_MICRO.37 R10.1 U$1.14 U$5.C U$7.C U$8.C U$11.SCL
SCL1: HAND_MICRO.55 R12.1 U$12.SCL
SCL2: HAND_MICRO1.37 R26.1 U$13.14 U$17.C U$18.C U$20.C U$23.SCL
SCL3: HAND_MICRO1.55 R28.1 U$24.SCL
SCL4: HAND_MICRO2.37 R42.1 U$25.14 U$29.C U$30.C U$32.C U$35.SCL
SCL5: HAND_MICRO2.55 R44.1 U$36.SCL
SCL6: HAND_MICRO3.37 R58.1 U$37.14 U$41.C U$42.C U$44.C U$47.SCL
SCL7: HAND_MICRO3.55 R60.1 U$48.SCL
SDA0: HAND_MICRO.38 R11.1 U$1.15 U$5.D U$7.D U$8.D U$11.SDA
SDA1: HAND_MICRO.56 R13.1 U$12.SDA
SDA2: HAND_MICRO1.38 R27.1 U$13.15 U$17.D U$18.D U$20.D U$23.SDA
SDA3: HAND_MICRO1.56 R29.1 U$24.SDA
SDA4: HAND_MICRO2.38 R43.1 U$25.15 U$29.D U$30.D U$32.D U$35.SDA
SDA5: HAND_MICRO2.56 R45.1 U$36.SDA
SDA6: HAND_MICRO3.38 R59.1 U$37.15 U$41.D U$42.D U$44.D U$47.SDA
SDA7: HAND_MICRO3.56 R61.1 U$48.SDA
THA1: THMB.16 THUMB_A.1
THA2: THMB.2 THUMB_A.2
THA3: THMB1.16 THUMB_A1.1
THA4: THMB1.2 THUMB_A1.2
THA5: THMB2.16 THUMB_A2.1
THA6: THMB2.2 THUMB_A2.2
THA7: THMB3.16 THUMB_A3.1
THA8: THMB3.2 THUMB_A3.2
THAENC1: HAND_MICRO.35 THUMB_A.5
THAENC2: HAND_MICRO.36 THUMB_A.4
THAENC3: HAND_MICRO1.36 THUMB_A1.4
THAENC4: HAND_MICRO1.35 THUMB_A1.5
THAENC5: HAND_MICRO2.36 THUMB_A2.4
THAENC6: HAND_MICRO2.35 THUMB_A2.5
THAENC7: HAND_MICRO3.36 THUMB_A3.4
THAENC8: HAND_MICRO3.35 THUMB_A3.5
THAISEN: HAND_MICRO.11 R4.2 THMB.1
THAISEN1: HAND_MICRO1.11 R20.2 THMB1.1
THAISEN2: HAND_MICRO2.11 R36.2 THMB2.1
THAISEN3: HAND_MICRO3.11 R52.2 THMB3.1
THAPWM1: HAND_MICRO.41 THMB.14
THAPWM2: HAND_MICRO.42 THMB.13
THAPWM3: HAND_MICRO1.42 THMB1.13
THAPWM4: HAND_MICRO1.41 THMB1.14
THAPWM5: HAND_MICRO2.42 THMB2.13
THAPWM6: HAND_MICRO2.41 THMB2.14
THAPWM7: HAND_MICRO3.42 THMB3.13
THAPWM8: HAND_MICRO3.41 THMB3.14
THB1: THMB.5 THUMB_B.2
THB2: THMB.3 THUMB_B.1
THB3: THMB1.3 THUMB_B1.1
THB4: THMB1.5 THUMB_B1.2
THB5: THMB2.3 THUMB_B2.1
THB6: THMB2.5 THUMB_B2.2
THB7: THMB3.3 THUMB_B3.1
THB8: THMB3.5 THUMB_B3.2
THBENC1: HAND_MICRO.51 THUMB_B.5
THBENC2: HAND_MICRO.50 THUMB_B.4
THBENC3: HAND_MICRO1.50 THUMB_B1.4
THBENC4: HAND_MICRO1.51 THUMB_B1.5
THBENC5: HAND_MICRO2.50 THUMB_B2.4
THBENC6: HAND_MICRO2.51 THUMB_B2.5
THBENC7: HAND_MICRO3.50 THUMB_B3.4
THBENC8: HAND_MICRO3.51 THUMB_B3.5
THBISEN: HAND_MICRO.12 R5.2 THMB.4
THBISEN1: HAND_MICRO1.12 R21.2 THMB1.4
THBISEN2: HAND_MICRO2.12 R37.2 THMB2.4
THBISEN3: HAND_MICRO3.12 R53.2 THMB3.4
THBPWM1: HAND_MICRO.45 THMB.7
THBPWM2: HAND_MICRO.44 THMB.8
THBPWM3: HAND_MICRO1.44 THMB1.8
THBPWM4: HAND_MICRO1.45 THMB1.7
THBPWM5: HAND_MICRO2.44 THMB2.8
THBPWM6: HAND_MICRO2.45 THMB2.7
THBPWM7: HAND_MICRO3.44 THMB3.8
THBPWM8: HAND_MICRO3.45 THMB3.7
USB_D1_N [USB]: D-.P$1 R1.1 USB.2
USB_D1_N1 [USB]: D-1.P$1 R17.1 USB1.2
USB_D1_N2 [USB]: D-2.P$1 R33.1 USB2.2
USB_D1_N3 [USB]: D-3.P$1 R49.1 USB3.2
USB_D1_P [USB]: D+.P$1 R2.1 USB.3
USB_D1_P1 [USB]: D+1.P$1 R18.1 USB1.3
USB_D1_P2 [USB]: D+2.P$1 R34.1 USB2.3
USB_D1_P3 [USB]: D+3.P$1 R50.1 USB3.3
USB_D2_N [USB]: HAND_MICRO.6 R1.2
USB_D2_N1 [USB]: HAND_MICRO1.6 R17.2
USB_D2_N2 [USB]: HAND_MICRO2.6 R33.2
USB_D2_N3 [USB]: HAND_MICRO3.6 R49.2
USB_D2_P [USB]: HAND_MICRO.5 R2.2
USB_D2_P1 [USB]: HAND_MICRO1.5 R18.2
USB_D2_P2 [USB]: HAND_MICRO2.5 R34.2
USB_D2_P3 [USB]: HAND_MICRO3.5 R50.2
VIN: U$2.2 U$10.B
VIN1: U$16.2 U$22.B
VIN2: U$28.2 U$34.B
VIN3: U$40.2 U$46.B

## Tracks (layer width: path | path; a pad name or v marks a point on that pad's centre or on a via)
+3V1  (via drill 0.38, 0.39)  (1 unrouted)
  Top 0.254: THUMB_A1.3 31.7,120.04 32.64,120.04 33.17,119.51 33.17,118.29 34.34,116.15 v34.44,114.83 | THUMB_B1.3 30.88,107.47 32.97,108.2 v33.63,110.16 | C32.1 57.13,108.31 57.02,108.31 56.59,108.66 HAND_MICRO1.21 53.59,108.66 52.73,109.42 52.3,109.86 v51.71,109.86 | 47.12,104.65 HAND_MICRO1.3 47.13,103.21 v46.86,102.95 | v49.55,106.38 49.13,106.14 HAND_MICRO1.7 49.13,103.58 49.02,103.48 | PINKY1.3 54.63,89.7 | 54.63,91.14 v54.57,91.2 | RING1.3 41.63,83.7 v41.66,84.94 | C33.1 45.73,101.81 | 49.02,103.48 48.84,103.3 v48.44,103.3 | MIDDLE1.3 25.7,82.73 v25.7,84.15 | INDEX1.3 12.83,81.76 v12.83,82.96 | HAND_MICRO1.8 49.63,103.76 49.62,103.71 49.39,103.48 49.02,103.48 | HAND_MICRO1.48 46.13,115.14 47.65,113.61 50.47,113.61 52.25,113.13 53.12,113.17 v53.09,113.15 | HAND_MICRO1.48 46.12,116.28 45.07,117.33 45.07,118.11 C35.1 | v59.91,113.56 59.74,113.56 59.04,112.86 58.48,112.86 C34.1 58.34,112.8 57.48,112.8 57.12,113.16 HAND_MICRO1.30 | v63.01,114.22 62.85,114.07 BOOTLOADER1.1 | HAND_MICRO1.48 44.83,116.16 v43.95,115.29 | U$13.1 31.37,88.21 | 31.37,88.21 31.37,88.9 | 31.37,88.9 31.37,89.51 U$13.3 34.35,89.51 C38.1 | U$13.2 32.37,88.9 31.37,88.9 | U$13.16 27.71,88.21 v27.81,88.21 | v31.09,88.21 31.37,88.21
  Top 0.762: 54.63,89.7 54.63,91.14 | v54.57,91.2 45.73,100.04 C33.1 | 45.73,101.81 45.9,102.18 46.66,102.95 v46.86,102.95
  Top 1.016: v63.01,114.22 62.36,115.41 61.8,116.53 60.05,117.45 60.05,120.22 59.46,121.36 57.68,121.36 55.31,123.18 R26.2 R27.2 | 49.4,123.22 48.44,123.22 v47.27,122.05 | C37.1 57.54,124.83 v54.28,123.6 54.3,123.27 53.57,123.22
  Route2 0.254: v33.63,110.16 v34.44,114.83 34.85,114.43 42.86,114.43 43.6,115.29 v43.95,115.29 | v54.57,91.2 54.57,89.85 47.09,82.37 42.96,82.37 RING1.3 v41.66,84.94 | v25.7,84.15 24.61,81.66 18.77,81.66 17.32,80.34 13.74,80.64 v12.83,82.96 | v27.81,88.21 v31.09,88.21
  Bottom 0.254: 50.94,108.33 U$15.1 51.02,108.97 51.02,109.16 | 47.22,103.3 v46.86,102.95 | R29.2 49.74,109.59 R28.2 | v41.66,84.94 41.66,83.29 40.77,82.4 32.46,82.4 31.19,80.39 28.27,80.39 | 28.27,80.39 27.56,81.69 25.7,83.54 v25.7,84.15 26.62,85.06 29.52,85.06 31.09,86.64 v31.09,88.21 | U$17.V 32.54,77.57 28.27,80.39 | U$20.V 8.89,79.02 v12.83,82.96
  Bottom 0.762: v51.71,109.86 51.71,111.4
  Bottom 1.016: U$15.1 50.47,108.51 49.45,107.49 49.45,104.72 47.98,103.25 | v48.44,103.3 47.22,103.3 | v51.71,109.86 51.02,109.16 | v63.01,114.22 60.57,114.22 v59.91,113.56 59.63,113.41 53.87,113.41 v53.09,113.15 51.71,111.4 | R29.2 50.34,108.97 51.02,108.97 | U$21.3 56.38,125.92 55.14,125.91 54.28,125.04 v54.28,123.6 | v43.95,115.29 43.97,115.3 44.76,116.56 47.27,119.18 v47.27,122.05
  pour Route2 (isolate 0.508): 48.06,77.17 47.75,83.34 67.18,84.33 65.15,125.58 62.74,128.24 24.49,128.24 24.61,125.7 24.89,124.59 25.22,123.77 25.58,122.89 26.16,120.62 26.47,118.26 26.49,116.1 26.39,115.52 26.24,114.43 25.58,110.62 25.04,107.24 24.74,106.71 24.51,106.07 23.27,104.27 22.25,103.17 21.01,102.18 19.56,101.27 17.68,100.43 14.58,99.54 11.4,98.58 5.66,96.72 4.42,70.79 17.35,70.1 17.4,75.69 41.86,81.66
+3V2  (via drill 0.38, 0.39)  (1 unrouted)
  Top 0.254: THUMB_A2.3 106.56,52.88 107.49,52.88 108.03,52.35 108.03,51.13 109.19,49 v109.3,47.68 | THUMB_B2.3 105.74,40.31 107.82,41.05 v108.48,43 | C51.1 131.99,41.15 131.88,41.15 131.44,41.51 HAND_MICRO2.21 128.45,41.51 127.58,42.27 127.15,42.7 v126.57,42.7 | 121.97,37.5 HAND_MICRO2.3 121.98,36.05 v121.72,35.79 | v124.41,39.22 123.98,38.99 HAND_MICRO2.7 123.98,36.43 123.88,36.32 | PINKY2.3 129.49,22.54 | 129.49,23.98 v129.43,24.04 | RING2.3 116.48,16.55 v116.51,17.78 | C52.1 120.58,34.65 | 123.88,36.32 123.7,36.14 v123.29,36.14 | MIDDLE2.3 100.56,15.57 v100.56,16.99 | INDEX2.3 87.68,14.61 v87.68,15.8 | HAND_MICRO2.8 124.48,36.61 124.47,36.55 124.24,36.32 123.88,36.32 | HAND_MICRO2.48 120.98,47.98 122.5,46.46 125.32,46.46 127.1,45.97 127.98,46.01 v127.95,45.99 | HAND_MICRO2.48 120.98,49.13 119.93,50.18 119.93,50.95 C54.1 | v134.76,46.41 134.59,46.41 133.9,45.71 133.33,45.71 C53.1 133.19,45.64 132.33,45.64 131.97,46.01 HAND_MICRO2.30 | v137.86,47.07 137.71,46.91 BOOTLOADER2.1 | HAND_MICRO2.48 119.68,49.01 v118.81,48.13 | U$25.1 106.22,21.05 106.22,21.06 | 106.22,21.06 106.22,21.74 | 106.22,21.74 106.22,22.35 U$25.3 109.21,22.35 C57.1 | U$25.2 107.23,21.74 106.22,21.74 | U$25.16 102.56,21.05 v102.67,21.06 | v105.94,21.06 106.22,21.06
  Top 0.762: 129.49,22.54 129.49,23.98 | v129.43,24.04 120.58,32.89 C52.1 | 120.58,34.65 120.75,35.03 121.51,35.79 v121.72,35.79
  Top 1.016: v137.86,47.07 137.21,48.25 136.65,49.38 134.9,50.29 134.9,53.06 134.31,54.2 132.54,54.2 130.16,56.02 R42.2 R43.2 | 124.26,56.06 123.29,56.06 v122.12,54.89 | C56.1 132.4,57.67 v129.13,56.44 129.16,56.11 128.42,56.06
  Route2 0.254: v108.48,43 v109.3,47.68 109.7,47.27 117.72,47.27 118.45,48.13 v118.81,48.13 | v129.43,24.04 129.43,22.7 121.94,15.21 117.82,15.21 RING2.3 v116.51,17.78 | v100.56,16.99 99.47,14.5 93.62,14.5 92.18,13.18 88.59,13.49 v87.68,15.8 | v102.67,21.06 v105.94,21.06
  Bottom 0.254: 125.79,41.17 U$27.1 125.87,41.81 125.87,42 | 122.07,36.14 v121.72,35.79 | R45.2 124.6,42.43 R44.2 | v116.51,17.78 116.51,16.13 115.62,15.24 107.31,15.24 106.05,13.23 103.12,13.23 | 103.12,13.23 102.41,14.53 100.56,16.38 v100.56,16.99 101.47,17.91 104.37,17.91 105.94,19.48 v105.94,21.06 | U$29.V 107.39,10.41 103.12,13.23 | U$32.V 83.74,11.86 v87.68,15.8
  Bottom 0.762: v126.57,42.7 126.57,44.25
  Bottom 1.016: U$27.1 125.32,41.35 124.31,40.34 124.31,37.57 122.83,36.09 | v123.29,36.14 122.07,36.14 | v126.57,42.7 125.87,42 | v137.86,47.07 135.42,47.07 v134.76,46.41 134.48,46.25 128.73,46.25 v127.95,45.99 126.57,44.25 | R45.2 125.2,41.81 125.87,41.81 | U$33.3 131.23,58.76 130,58.75 129.13,57.89 v129.13,56.44 | v118.81,48.13 118.82,48.15 119.61,49.4 122.12,52.02 v122.12,54.89
  pour Route2 (isolate 0.508): 122.91,10.01 122.61,16.18 142.04,17.17 140,58.42 137.59,61.09 99.34,61.09 99.47,58.55 99.75,57.43 100.08,56.62 100.43,55.73 101.02,53.47 101.32,51.1 101.35,48.95 101.24,48.36 101.09,47.27 100.43,43.46 99.9,40.08 99.59,39.55 99.36,38.91 98.12,37.11 97.1,36.02 95.86,35.03 94.41,34.11 92.53,33.27 89.43,32.38 86.26,31.42 80.52,29.57 79.27,3.63 92.2,2.95 92.25,8.53 116.71,14.5
+3V3  (via drill 0.38, 0.39)  (1 unrouted)
  Top 0.254: THUMB_A.3 40.05,13.59 39.12,13.59 38.58,14.12 38.58,15.34 37.41,17.48 v37.31,18.8 | THUMB_B.3 40.87,26.16 38.79,25.43 v38.12,23.47 | C13.1 14.62,25.32 14.73,25.32 15.17,24.97 HAND_MICRO.21 18.16,24.97 19.02,24.21 19.46,23.77 v20.04,23.77 | HAND_MICRO.3 24.63,30.42 v24.89,30.68 | v22.2,27.25 22.63,27.49 HAND_MICRO.7 22.63,30.05 22.73,30.15 | PINKY.3 17.12,43.93 | 17.12,42.49 v17.18,42.43 | RING.3 30.12,49.92 v30.1,48.69 | C14.1 26.03,31.82 | 22.73,30.15 22.91,30.33 v23.32,30.33 | MIDDLE.3 46.05,50.9 v46.05,49.48 | INDEX.3 58.93,51.87 v58.93,50.67 | HAND_MICRO.8 22.13,29.87 22.14,29.92 22.36,30.15 22.73,30.15 | HAND_MICRO.48 25.63,18.49 24.11,20.02 21.29,20.02 19.51,20.5 18.63,20.46 v18.66,20.48 | HAND_MICRO.48 25.63,17.34 26.68,16.29 26.68,15.53 C16.1 | v11.85,20.07 12.01,20.07 12.71,20.77 13.28,20.77 C15.1 13.42,20.83 14.28,20.83 14.64,20.47 HAND_MICRO.30 | v8.75,19.41 8.9,19.56 BOOTLOADER.1 | HAND_MICRO.48 26.93,17.47 v27.8,18.34 | U$1.1 40.39,45.42 40.39,45.41 | 40.39,45.41 40.39,44.73 | 40.39,44.73 40.39,44.12 U$1.3 37.4,44.12 C19.1 | U$1.2 39.38,44.73 40.39,44.73 | U$1.16 44.04,45.42 v43.94,45.41 | v40.66,45.41 40.39,45.41
  Top 0.762: 17.12,43.93 17.12,42.49 | v17.18,42.43 26.03,33.59 C14.1 | 26.03,31.82 25.86,31.45 25.09,30.68 v24.89,30.68
  Top 1.016: v8.75,19.41 9.4,18.22 9.96,17.09 11.71,16.18 11.71,13.41 12.29,12.27 14.07,12.27 16.45,10.45 R10.2 R11.2 | 22.35,10.41 23.32,10.41 v24.49,11.58 | C18.1 14.21,8.8 v17.48,10.03 17.45,10.36 18.19,10.41
  Route2 0.254: v38.12,23.47 v37.31,18.8 36.91,19.2 28.89,19.2 28.16,18.34 v27.8,18.34 | v17.18,42.43 17.18,43.78 24.66,51.26 28.79,51.26 RING.3 v30.1,48.69 | v46.05,49.48 47.14,51.97 52.98,51.97 54.43,53.29 58.01,52.98 v58.93,50.67 | v43.94,45.41 v40.66,45.41
  Bottom 0.254: 20.82,25.3 U$4.1 20.74,24.66 20.74,24.47 | 24.54,30.33 v24.89,30.68 | R13.2 22.01,24.04 R12.2 | v30.1,48.69 30.1,50.34 30.99,51.23 39.29,51.23 40.56,53.24 43.48,53.24 | 43.48,53.24 44.2,51.94 46.05,50.09 v46.05,49.48 45.14,48.56 42.24,48.56 40.66,46.99 v40.66,45.41 | U$5.V 39.22,56.06 43.48,53.24 | U$8.V 62.87,54.61 v58.93,50.67
  Bottom 0.762: v20.04,23.77 20.04,22.23
  Bottom 1.016: U$4.1 21.29,25.12 22.3,26.14 22.3,28.91 23.77,30.38 | v23.32,30.33 24.54,30.33 | v20.04,23.77 20.74,24.47 | v8.75,19.41 11.19,19.41 v11.85,20.07 12.13,20.22 17.88,20.22 v18.66,20.48 20.04,22.23 | R13.2 21.41,24.66 20.74,24.66 | U$9.3 15.38,7.71 16.61,7.72 17.48,8.59 v17.48,10.03 | v27.8,18.34 27.79,18.33 27,17.07 24.49,14.45 v24.49,11.58
  pour Route2 (isolate 0.508): 23.7,56.46 24,50.29 4.57,49.3 6.6,8.05 9.02,5.38 47.27,5.38 47.14,7.92 46.86,9.04 46.53,9.86 46.18,10.74 45.59,13 45.29,15.37 45.26,17.53 45.36,18.11 45.52,19.2 46.18,23.01 46.71,26.39 47.02,26.92 47.24,27.56 48.49,29.36 49.5,30.45 50.75,31.45 52.2,32.36 54.08,33.2 57.18,34.09 60.35,35.05 66.09,36.91 67.34,62.84 54.41,63.53 54.36,57.94 29.9,51.97
+3V4  (via drill 0.38, 0.39)  (1 unrouted)
  Top 0.254: THUMB_A3.3 115.03,80.59 114.1,80.59 113.56,81.13 113.56,82.35 112.39,84.48 v112.29,85.8 | THUMB_B3.3 115.85,93.17 113.77,92.43 v113.11,90.47 | C70.1 89.6,92.33 89.71,92.33 90.15,91.97 HAND_MICRO3.21 93.14,91.97 94,91.21 94.44,90.78 v95.02,90.78 | HAND_MICRO3.3 99.61,97.42 v99.87,97.69 | v97.18,94.26 97.61,94.49 HAND_MICRO3.7 97.61,97.05 97.71,97.16 | PINKY3.3 92.1,110.93 | 92.1,109.5 v92.16,109.44 | RING3.3 105.11,116.93 v105.08,115.7 | C71.1 101.01,98.83 | 97.71,97.16 97.89,97.33 v98.3,97.33 | MIDDLE3.3 121.03,117.91 v121.03,116.48 | INDEX3.3 133.91,118.87 v133.91,117.68 | HAND_MICRO3.8 97.11,96.87 97.12,96.93 97.35,97.16 97.71,97.16 | HAND_MICRO3.48 100.61,85.5 99.08,87.02 96.27,87.02 94.49,87.5 93.61,87.47 v93.64,87.49 v93.64,87.48 | HAND_MICRO3.48 100.61,84.35 101.66,83.3 101.66,82.53 C73.1 | v86.83,87.07 87,87.07 87.69,87.77 88.26,87.77 C72.1 88.4,87.83 89.26,87.83 89.62,87.47 HAND_MICRO3.30 | v83.73,86.41 83.88,86.56 BOOTLOADER3.1 | HAND_MICRO3.48 101.91,84.47 v102.78,85.34 | U$37.1 115.37,112.43 115.37,112.42 | 115.37,112.42 115.37,111.73 | 115.37,111.73 115.37,111.13 U$37.3 112.38,111.13 C76.1 | U$37.2 114.36,111.73 115.37,111.73 | U$37.16 119.02,112.43 v118.92,112.42 | v115.65,112.42 115.37,112.42
  Top 0.762: 92.1,110.93 92.1,109.5 | v92.16,109.44 101.01,100.59 C71.1 | 101.01,98.83 100.84,98.45 100.08,97.69 v99.87,97.69
  Top 1.016: v83.73,86.41 84.38,85.23 84.94,84.1 86.69,83.19 86.69,80.42 87.27,79.27 89.05,79.27 91.43,77.46 R58.2 R59.2 | 97.33,77.42 98.3,77.42 v99.47,78.59 | C75.1 89.19,75.81 v92.46,77.04 92.43,77.37 93.17,77.42
  Route2 0.254: v113.11,90.47 v112.29,85.8 111.89,86.21 103.87,86.21 103.14,85.34 v102.78,85.34 | v92.16,109.44 92.16,110.78 99.64,118.26 103.77,118.26 RING3.3 v105.08,115.7 | v121.03,116.48 122.12,118.97 127.97,118.97 129.41,120.29 132.99,119.99 v133.91,117.68 | v118.92,112.42 v115.65,112.42
  Bottom 0.254: 95.8,92.3 U$39.1 95.72,91.67 95.72,91.47 | 99.52,97.33 v99.87,97.69 | R61.2 96.99,91.05 R60.2 | v105.08,115.7 105.08,117.35 105.97,118.24 114.28,118.24 115.55,120.24 118.47,120.24 | 118.47,120.24 119.18,118.95 121.03,117.09 v121.03,116.48 120.12,115.57 117.22,115.57 115.65,114 v115.65,112.42 | U$41.V 114.2,123.06 118.47,120.24 | U$44.V 137.85,121.61 v133.91,117.68
  Bottom 0.762: v95.02,90.78 95.02,89.23
  Bottom 1.016: U$39.1 96.27,92.13 97.28,93.14 97.28,95.91 98.75,97.38 | v98.3,97.33 99.52,97.33 | v95.02,90.78 95.72,91.47 | v83.73,86.41 86.17,86.41 v86.83,87.07 87.11,87.22 92.86,87.22 v93.64,87.48 95.02,89.23 | R61.2 96.39,91.67 95.72,91.67 | U$45.3 90.36,74.71 91.59,74.73 92.46,75.59 v92.46,77.04 | v102.78,85.34 102.77,85.33 101.98,84.07 99.47,81.46 v99.47,78.59
  pour Route2 (isolate 0.508): 98.68,123.47 98.98,117.3 79.55,116.31 81.58,75.06 84,72.39 122.25,72.39 122.12,74.93 121.84,76.05 121.51,76.86 121.16,77.75 120.57,80.01 120.27,82.37 120.24,84.53 120.35,85.12 120.5,86.21 121.16,90.02 121.69,93.4 122,93.93 122.22,94.56 123.47,96.37 124.49,97.46 125.73,98.45 127.18,99.36 129.06,100.2 132.16,101.09 135.33,102.06 141.07,103.91 142.32,129.84 129.39,130.53 129.34,124.94 104.88,118.97
+5V  (via drill 0.38, 0.39)
  Top 0.254: THMB.15 35.43,15.04 36.12,14.35 36.12,11.23 36.94,10.4 39.27,10.4 v40.68,8.99 | PKYRNG.15 27.05,45.32 27.36,45.62 34.58,45.62 34.85,45.35 34.85,40.62 34.09,39.85 C6.1 34.09,40.07 | 29.62,8.2 C9.1 30.01,7.27 v31.17,6.11 | 31.27,10.8 31.55,10.83 | INDMID.15 65.07,45.04 66.41,43.7 66.13,39.9 64.45,38.33 64.45,36.82 64.03,36.4 60.81,36.4 59.05,38.15
  Top 0.381: 31.55,10.83 31.55,11.48 THMB.10 | PKYRNG.10 30.95,40.89 31.22,40.7 | C6.1 | INDMID.10 60.55,41.05 60.35,41.02 | 59.09,38.97 58.88,38.76
  Top 0.762: 30.86,10.34 31.27,10.8 | 31.22,40.7 31.93,40.39 | 60.35,41.02 60.13,40.41
  Top 1.016: v13.28,10.95 11.88,10.95 C17.1
  Top 1.27: C4.2 C6.1 | C1.2 58.88,38.76 C3.1 | C9.1 29.22,8.19 C7.2 | 29.62,8.2 29.62,9.68 30.28,10.34 30.86,10.34 | 31.93,40.39 32.8,39.85 C6.1 | 60.13,40.41 59.26,39.38 59.09,38.97
  Top 1.524: C4.2 35.12,38.52 35.62,38.02 35.62,35.31 v35.6,35.28 | v56.63,35.4 58.26,35.4 59.05,36.88 59.05,38.15 59.05,38.58 58.88,38.76
  Top 1.905: 24.59,6.64 25.03,6.18 28.47,6.18 29.22,6.57 29.22,8.19
  Top 2.794: v24.57,7.7 24.59,7.92 24.59,6.64
  Bottom 0.254: v40.68,8.99 40.68,9.02 39.31,10.39 35.45,10.39 v31.17,6.11
  Bottom 1.016: v23.47,8.48 20.43,11.52 U$9.1 13.86,11.52 v13.28,10.95
  Bottom 1.524: 34.47,9.65 34.89,10.07 35.34,10.07 35.48,10.21 35.69,10.21 35.88,10.4 36.18,10.4 36.4,10.62 37.03,10.62 37.58,11.16 38.05,11.16
  Bottom 1.905: 33.08,9.27 33.47,9.65 34.47,9.65
  Bottom 2.794: v35.6,35.28 35.6,33.6 36.64,32.56 | 36.64,32.56 40.15,32.56 40.6,33.02 44.12,33.02 | 44.12,33.02 45.9,33.02 46.58,33.71 49.73,33.71 52.91,35.1 55.65,35.1 v56.63,35.4 | 36.64,32.56 36.6,32.52 | 43.27,25.59 43.27,15.49 | 43.27,15.49 43.27,15.34 | v24.57,7.7 33.1,7.71 33.08,7.72 33.08,9.27 | 38.05,11.16 42.38,15.49 43.27,15.49 | 42.76,26.1 44.12,27.46 44.12,33.02
  Bottom 3.81: U$2.3 40.6,37.82 40.6,33.02
  other vias: 41.76,35.23 39.41,36.28 57.35,36.44 39.37,34.34 35.56,33.9 55.26,35.74 55.63,34.19 58.23,35.13 25.93,6.82 25.3,8.7 23.42,7.12 24.54,6.35 27.95,6.59 29.45,6.55
  pour Top (isolate 0.406): 30.72,40.93 32.65,40.93 33.26,40.32 35.8,40.32 40.34,39.89 42.48,38.21 42.38,33.59 34.3,33.31 34.24,35.67 34.77,35.84 34.77,37.62 34.57,37.82 32.87,37.82 30.99,39.7 30.99,40.61 30.7,40.91
  pour Top (isolate 0.406): 60.63,41.5 60.63,39.83 60.26,39.46 60.26,35.9 58.53,34.44 55.09,33.55 54.5,33.97 54.13,35.56 54.74,36.35 55.99,37.38 57.86,37.52 57.86,40.08 58.76,40.98 60.01,40.98 60.53,41.5
  pour Top (isolate 0.406): 31.58,11.24 31.58,9.96 30.61,8.98 30.61,7.39 31.08,6.92 31.64,6.92 31.94,6.62 31.94,5.51 31.38,4.95 23.62,4.95 22.52,6.06 22.52,7.81 23.71,9 25.22,9 25.88,8.34 25.88,7.54 26.63,6.79 27.62,6.79 28.09,7.26 28.09,9.59 29.4,10.9 30.54,10.9 30.86,11.21 31.53,11.21 31.55,11.23
  pour Bottom (isolate 1.016, rank 2): 39.93,39.71 43.43,39.71 44.62,38.56 46.86,36.45 50.57,36.26 53.33,36.21 54.85,36.58 56.03,37.26 57.96,37.01 59.05,36.35 59.02,35.28 58.42,34.54 57.15,34.19 55.35,33.71 53.58,33.07 52.12,32.38 50.28,31.15 48.91,29.86 47.8,28.41 46.93,26.95 46.71,26.26 45.63,20.1 45.29,18.01 45.25,15.43 45.4,14.21 45.54,12.98 46.11,10.79 46.63,9.51 46.98,8.5 47.12,7.52 47.27,5.36 23.27,5.4 21.55,5.89 21.59,8.51 24.28,10.19 27.88,11.46 27.42,18.36 35.84,19.15 37.9,21.65 35.61,26.85 32.21,31.36 28.83,35.99 23.05,36.54 22,48.13 36.77,46.25
+5V1  (via drill 0.38, 0.39)
  Top 0.254: THMB1.15 36.33,118.59 35.64,119.28 35.64,122.4 34.81,123.23 32.49,123.23 v31.08,124.64 | PKYRNG1.15 44.7,88.31 44.4,88.01 37.17,88.01 36.91,88.28 36.91,93.02 37.67,93.78 C25.1 37.66,93.56 | 42.14,125.43 C28.1 41.75,126.36 v40.59,127.52 | 40.48,122.83 40.21,122.8 | INDMID1.15 6.69,88.59 5.35,89.93 5.63,93.73 7.3,95.3 7.3,96.81 7.72,97.23 10.95,97.23 12.7,95.48
  Top 0.381: 40.21,122.8 40.21,122.15 THMB1.10 | PKYRNG1.10 40.8,92.74 40.54,92.93 | C25.1 | INDMID1.10 11.2,92.58 11.4,92.61 | 12.66,94.66 12.88,94.88
  Top 0.762: 40.89,123.29 40.48,122.83 | 40.54,92.93 39.83,93.24 | 11.4,92.61 11.62,93.22
  Top 1.016: v58.47,122.68 59.88,122.68 C36.1
  Top 1.27: C23.2 C25.1 | C20.2 12.88,94.88 C22.1 | C28.1 42.53,125.44 C26.2 | 42.14,125.43 42.14,123.95 41.48,123.29 40.89,123.29 | 39.83,93.24 38.95,93.78 C25.1 | 11.62,93.22 12.5,94.25 12.66,94.66
  Top 1.524: C23.2 36.63,95.1 36.13,95.61 36.13,98.32 v36.16,98.35 | v15.13,98.23 13.5,98.23 12.7,96.75 12.7,95.48 12.7,95.05 12.88,94.88
  Top 1.905: 47.17,126.99 46.72,127.44 43.28,127.44 42.53,127.06 42.53,125.44
  Top 2.794: v47.18,125.93 47.17,125.7 47.17,126.99
  Bottom 0.254: v31.08,124.64 31.08,124.61 32.45,123.24 36.31,123.24 v40.59,127.52
  Bottom 1.016: v48.28,125.15 51.32,122.11 U$21.1 57.9,122.11 v58.47,122.68
  Bottom 1.524: 37.29,123.98 36.87,123.56 36.41,123.56 36.27,123.42 36.07,123.42 35.88,123.23 35.57,123.23 35.36,123.01 34.72,123.01 34.18,122.47 33.71,122.47
  Bottom 1.905: 38.67,124.36 38.29,123.98 37.29,123.98
  Bottom 2.794: v36.16,98.35 36.16,100.03 35.12,101.07 | 35.12,101.07 31.61,101.07 31.15,100.61 27.64,100.61 | 27.64,100.61 25.86,100.61 25.17,99.92 22.02,99.92 18.85,98.53 16.1,98.53 v15.13,98.23 | 35.12,101.07 35.15,101.11 | 28.49,108.04 28.49,118.14 | 28.49,118.14 28.49,118.29 | v47.18,125.93 38.66,125.92 38.67,125.91 38.67,124.36 | 33.71,122.47 29.38,118.14 28.49,118.14 | 28.99,107.53 27.64,106.17 27.64,100.61
  Bottom 3.81: U$16.3 31.15,95.81 31.15,100.61
  other vias: 30,98.4 32.35,97.35 14.4,97.19 32.38,99.29 36.2,99.73 16.5,97.89 16.13,99.44 13.53,98.5 45.82,126.81 46.46,124.93 48.34,126.5 47.22,127.28 43.8,127.04 42.3,127.08
  pour Top (isolate 0.406): 41.03,92.7 39.1,92.7 38.49,93.31 35.95,93.31 31.42,93.74 29.27,95.42 29.38,100.04 37.45,100.32 37.52,97.96 36.98,97.79 36.98,96.01 37.19,95.81 38.89,95.81 40.77,93.93 40.77,93.01 41.06,92.72
  pour Top (isolate 0.406): 11.13,92.13 11.13,93.8 11.49,94.17 11.49,97.73 13.22,99.19 16.66,100.08 17.26,99.66 17.63,98.07 17.02,97.28 15.76,96.25 13.89,96.11 13.89,93.55 12.99,92.65 11.75,92.65 11.23,92.13
  pour Top (isolate 0.406): 40.17,122.39 40.17,123.67 41.15,124.65 41.15,126.24 40.68,126.71 40.12,126.71 39.81,127.01 39.81,128.12 40.37,128.68 48.13,128.68 49.24,127.57 49.24,125.82 48.04,124.63 46.53,124.63 45.87,125.29 45.87,126.09 45.12,126.83 44.13,126.83 43.66,126.36 43.66,124.04 42.35,122.73 41.21,122.73 40.89,122.42 40.22,122.42 40.21,122.4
